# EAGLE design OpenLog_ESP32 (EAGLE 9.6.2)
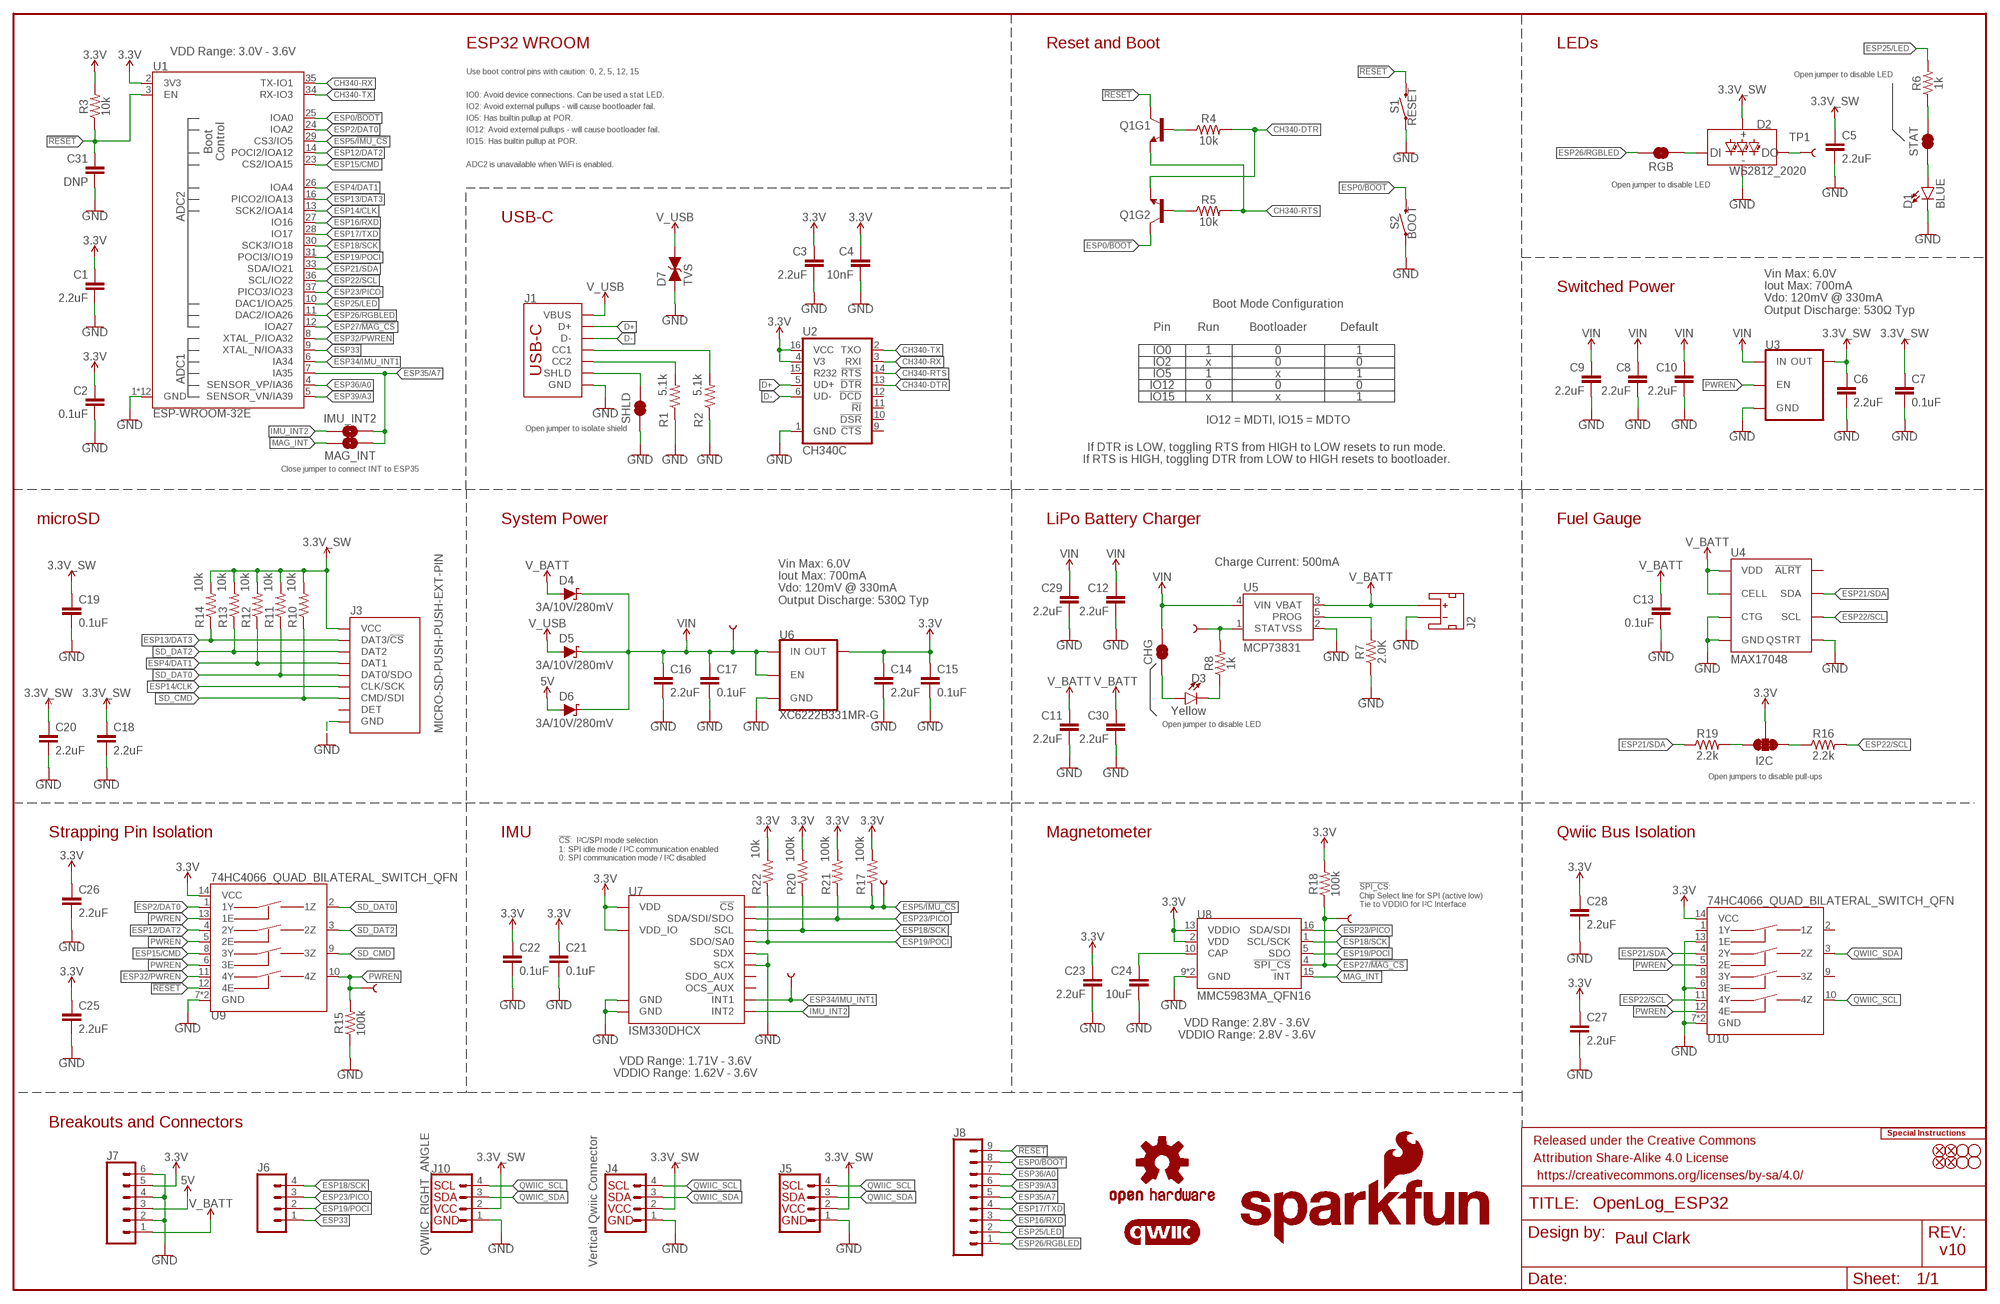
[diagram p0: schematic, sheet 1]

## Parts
C1  2.2uF  2.2UF-0402_TIGHT-10V-10%-X5R  [0402-TIGHT]
C2  0.1uF  0.1UF-0402T-6.3V-10%-X7R  [0402-TIGHT]
C3  2.2uF  2.2UF-0402_TIGHT-10V-10%-X5R  [0402-TIGHT]
C4  10nF  10NF-0402T-25V-10%-X7R-WE  [0402-TIGHT]
C5  2.2uF  2.2UF-0402_TIGHT-10V-10%-X5R  [0402-TIGHT]
C6  2.2uF  2.2UF-0402_TIGHT-10V-10%-X5R  [0402-TIGHT]
C7  0.1uF  0.1UF-0402T-6.3V-10%-X7R  [0402-TIGHT]
C8  2.2uF  2.2UF-0402_TIGHT-10V-10%-X5R  [0402-TIGHT]
C9  2.2uF  2.2UF-0402_TIGHT-10V-10%-X5R  [0402-TIGHT]
C10  2.2uF  2.2UF-0402_TIGHT-10V-10%-X5R  [0402-TIGHT]
C11  2.2uF  2.2UF-0402_TIGHT-10V-10%-X5R  [0402-TIGHT]
C12  2.2uF  2.2UF-0402_TIGHT-10V-10%-X5R  [0402-TIGHT]
C13  0.1uF  0.1UF-0402T-6.3V-10%-X7R  [0402-TIGHT]
C14  2.2uF  2.2UF-0402_TIGHT-10V-10%-X5R  [0402-TIGHT]
C15  0.1uF  0.1UF-0402T-6.3V-10%-X7R  [0402-TIGHT]
C16  2.2uF  2.2UF-0402_TIGHT-10V-10%-X5R  [0402-TIGHT]
C17  0.1uF  0.1UF-0402T-6.3V-10%-X7R  [0402-TIGHT]
C18  2.2uF  2.2UF-0402_TIGHT-10V-10%-X5R  [0402-TIGHT]
C19  0.1uF  0.1UF-0402T-6.3V-10%-X7R  [0402-TIGHT]
C20  2.2uF  2.2UF-0402_TIGHT-10V-10%-X5R  [0402-TIGHT]
C21  0.1uF  0.1UF-0402T-6.3V-10%-X7R  [0402-TIGHT]
C22  0.1uF  0.1UF-0402T-6.3V-10%-X7R  [0402-TIGHT]
C23  2.2uF  2.2UF-0402_TIGHT-10V-10%-X5R  [0402-TIGHT]
C24  10uF  10UF-0402T-6.3V-20%  [0402-TIGHT]
C25  2.2uF  2.2UF-0402_TIGHT-10V-10%-X5R  [0402-TIGHT]
C26  2.2uF  2.2UF-0402_TIGHT-10V-10%-X5R  [0402-TIGHT]
C27  2.2uF  2.2UF-0402_TIGHT-10V-10%-X5R  [0402-TIGHT]
C28  2.2uF  2.2UF-0402_TIGHT-10V-10%-X5R  [0402-TIGHT]
C29  2.2uF  2.2UF-0402_TIGHT-10V-10%-X5R  [0402-TIGHT]
C30  2.2uF  2.2UF-0402_TIGHT-10V-10%-X5R  [0402-TIGHT]
C31  DNP  DNP-0402-TIGHT_NO_CREAM  [0402-TIGHT_NO_CREAM]
CHG  JUMPER-SMT_2_NC_TRACE_SILK  [SMT-JUMPER_2_NC_TRACE_SILK]
D1  BLUE  LED-BLUE0603  [LED-0603]
D2  WS2812_2020  [WS2812-2020]
D3  Yellow  LED-YELLOW0603  [LED-0603]
D4  3A/10V/280mV  DIODE-SCHOTTKY-BAT60A  [SOD-323]
D5  3A/10V/280mV  DIODE-SCHOTTKY-BAT60A  [SOD-323]
D6  3A/10V/280mV  DIODE-SCHOTTKY-BAT60A  [SOD-323]
D7  TVS  DIODE_TVS  [0603]
FD1  FIDUCIAL1X2  [FIDUCIAL-1X2]
FD2  FIDUCIAL1X2  [FIDUCIAL-1X2]
FD3  FIDUCIAL1X2  [FIDUCIAL-1X2]
FD4  FIDUCIAL1X2  [FIDUCIAL-1X2]
FRAME1  FRAME-LEDGER  [CREATIVE_COMMONS]
H1  STAND-OFFTIGHT  [STAND-OFF-TIGHT]
H2  STAND-OFFTIGHT  [STAND-OFF-TIGHT]
H3  STAND-OFFTIGHT  [STAND-OFF-TIGHT]
H4  STAND-OFFTIGHT  [STAND-OFF-TIGHT]
I2C  JUMPER-SMT_3_2-NC_TRACE_SILK  [SMT-JUMPER_3_2-NC_TRACE_SILK]
IMU_!CS!  TEST-POINT3X5  [PAD.03X.05]
IMU_INT1  TEST-POINT3X5  [PAD.03X.05]
IMU_INT2  JUMPER-SMT_2_NO_SILK  [SMT-JUMPER_2_NO_SILK]
J1  USB_C_4-LAYER_PADS  [USB-C-16P_4LAYER-PADS]
J2  JST_2MM_MALE  [JST-2-SMD]
J3  MICRO-SD-PUSH-PUSH-EXT-PIN  [MICROSD-EXTERNALPIN]
J4  Vertical Qwiic Connector  QWIIC_CONNECTOR  [JST04_1MM_VERT]
J5  I2C_STANDARD_NO_SILK  [1X04_NO_SILK]
J6  CONN_041X04_NO_SILK_NO_POP  [1X04_NO_SILK]
J7  CONN_06NO_SILK_NO_POP  [1X06_NO_SILK]
J8  CONN_09NO_SILK  [1X09_NO_SILK]
J10  QWIIC_RIGHT_ANGLE  QWIIC_CONNECTORJS-1MM  [JST04_1MM_RA]
LOGO1  SPECIAL_INSTRUCTIONS-ORDERING  [ORDERING_INSTRUCTIONS]
LOGO3  QWIIC_LOGO_6MM  [QWIIC_6MM]
LOGO4  OSHW-LOGOS  [OSHW-LOGO-S]
LOGO5  SFE_LOGO_NAME.2_INCH  [SFE_LOGO_NAME_.2]
LOGO6  SFE_LOGO_FLAME.2_INCH  [SFE_LOGO_FLAME_.2]
MAG_!CS!  TEST-POINT3X5  [PAD.03X.05]
MAG_INT  JUMPER-SMT_2_NO_SILK  [SMT-JUMPER_2_NO_SILK]
PWREN  TEST-POINT3X5  [PAD.03X.05]
Q1  TRANS_NPN_DUAL-MBT3904DW1T1  [SC70-6]
R1  5.1k  5.1KOHM-0402T-1/16W-1%  [0402-TIGHT]
R2  5.1k  5.1KOHM-0402T-1/16W-1%  [0402-TIGHT]
R3  10k  10KOHM-0402T-1/16W-1%  [0402-TIGHT]
R4  10k  10KOHM-0402T-1/16W-1%  [0402-TIGHT]
R5  10k  10KOHM-0402T-1/16W-1%  [0402-TIGHT]
R6  1k  1KOHM-0402T-1/16W-1%  [0402-TIGHT]
R7  2.0K  2.0KOHM-0402T-1/16W-1%  [0402-TIGHT]
R8  1k  1KOHM-0402T-1/16W-1%  [0402-TIGHT]
R10  10k  10KOHM-0402T-1/16W-1%  [0402-TIGHT]
R11  10k  10KOHM-0402T-1/16W-1%  [0402-TIGHT]
R12  10k  10KOHM-0402T-1/16W-1%  [0402-TIGHT]
R13  10k  10KOHM-0402T-1/16W-1%  [0402-TIGHT]
R14  10k  10KOHM-0402T-1/16W-1%  [0402-TIGHT]
R15  100k  100KOHM-0402T-1/16W-1%  [0402-TIGHT]
R16  2.2k  2.2KOHM-0402T-1/16W-1%  [0402-TIGHT]
R17  100k  100KOHM-0402T-1/16W-1%  [0402-TIGHT]
R18  100k  100KOHM-0402T-1/16W-1%  [0402-TIGHT]
R19  2.2k  2.2KOHM-0402T-1/16W-1%  [0402-TIGHT]
R20  100k  100KOHM-0402T-1/16W-1%  [0402-TIGHT]
R21  100k  100KOHM-0402T-1/16W-1%  [0402-TIGHT]
R22  10k  10KOHM-0402T-1/16W-1%  [0402-TIGHT]
RGB  JUMPER-SMT_2_NC_TRACE_SILK  [SMT-JUMPER_2_NC_TRACE_SILK]
S1  RESET  MOMENTARY-SWITCH-SPST-SMD-RIGHT-ANGLE  [TACTILE_SWITCH_SMD_RIGHT_ANGLE]
S2  BOOT  MOMENTARY-SWITCH-SPST-SMD-RIGHT-ANGLE  [TACTILE_SWITCH_SMD_RIGHT_ANGLE]
SHLD  JUMPER-SMT_2_NC_TRACE_SILK  [SMT-JUMPER_2_NC_TRACE_SILK]
STAT  JUMPER-SMT_2_NC_TRACE_SILK  [SMT-JUMPER_2_NC_TRACE_SILK]
TP1  TEST-POINT3X5  [PAD.03X.05]
U1  ESP-WROOM-32E  ESP-WROOM-3232D-NARROW  [ESP-WROOM-32D-NARROW]
U2  CH340C  [SO016]
U3  XC6222B331MR-G  [SOT23-5]
U4  MAX17048  MAX17048DFN8  [DFN-8]
U5  MCP73831  [SOT23-5]
U6  XC6222B331MR-G  [SOT23-5]
U7  ISM330DHCX  [LGA-14L]
U8  MMC5983MA_QFN16  [LGA-16-3X3MM-4X4PINS]
U9  74HC4066_QUAD_BILATERAL_SWITCH_QFN  [14-QFN]
U10  74HC4066_QUAD_BILATERAL_SWITCH_QFN  [14-QFN]
VIN  TEST-POINT3X5  [PAD.03X.05]
VIN1  TEST-POINT3X5  [PAD.03X.05]

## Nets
3.3V: C1.1 C2.1 C3.1 C4.1 C14.1 C15.1 C21.1 C22.1 C23.1 C25.1 C26.1 C27.1 C28.1 I2C.2 J7.5 R3.2 R17.2 R18.2 R20.2 R21.2 R22.2 U1.2(3V3) U2.4(V3) U2.16(VCC) U6.5(OUT) U7.P5(VDD_IO) U7.P8(VDD) U8.2(VDD) U8.13(VDDIO) U9.14(VCC) U10.14(VCC)
3.3V_SW: C5.1 C6.1 C7.1 C18.1 C19.1 C20.1 D2.VCC J3.4(VCC) J4.2 J5.2 J10.2 R10.2 R11.2 R12.2 R13.2 R14.2 U3.5(OUT)
5V: D6.A J7.3
!RESET!: C31.1 J8.9 Q1.3(C) R3.1 S1.2 U1.3(EN) U9.12(4E)
CAP: C24.1 U8.10(CAP)
CH340-DTR: Q1.1(E) R4.2 U2.13(!DTR)
CH340-RTS: Q1.4(E) R5.2 U2.14(!RTS)
CH340-RX: U1.35(TX-IO1) U2.3(RXI)
CH340-TX: U1.34(RX-IO3) U2.2(TXO)
D+: J1.A6(D+) J1.B6(D+) U2.5(UD+)
D-: J1.A7(D-) J1.B7(D-) U2.6(UD-)
ESP0/!BOOT!: J8.8 Q1.6(C) S2.2 U1.25(IOA0)
ESP2/DAT0: U1.24(IOA2) U9.1(1Y)
ESP4/DAT1: J3.8(DAT1) R12.1 U1.26(IOA4)
ESP5/!IMU_CS!: IMU_!CS!.1 R17.1 U1.29(CS3/IO5) U7.P12(!CS!)
ESP12/DAT2: U1.14(POCI2/IOA12) U9.4(2Y)
ESP13/DAT3: J3.2(DAT3/!CS!) R14.1 U1.16(PICO2/IOA13)
ESP14/CLK: J3.5(CLK/SCK) U1.13(SCK2/IOA14)
ESP15/CMD: U1.23(CS2/IOA15) U9.8(3Y)
ESP16/RXD: J8.3 U1.27(IO16)
ESP17/TXD: J8.4 U1.28(IO17)
ESP18/SCK: J6.4 R20.1 U1.30(SCK3/IO18) U7.P13(SCL) U8.1(SCL/SCK)
ESP19/POCI: J6.2 R22.1 U1.31(POCI3/IO19) U7.P1(SDO/SA0) U8.5(SDO)
ESP21/SDA: R19.1 U1.33(SDA/IO21) U4.8(SDA) U10.4(2Y)
ESP22/SCL: R16.2 U1.36(SCL/IO22) U4.7(SCL) U10.11(4Y)
ESP23/PICO: J6.3 R21.1 U1.37(PICO3/IO23) U7.P14(SDA/SDI/SDO) U8.16(SDA/SDI)
ESP25/LED: J8.2 R6.2 U1.10(DAC1/IOA25)
ESP26/RGBLED: J8.1 RGB.2 U1.11(DAC2/IOA26)
ESP27/!MAG_CS!: MAG_!CS!.1 R18.1 U1.12(IOA27) U8.4(!SPI_CS!)
ESP32/PWREN: U1.8(XTAL_P/IOA32) U9.11(4Y)
ESP33: J6.1 U1.9(XTAL_N/IOA33)
ESP34/IMU_INT1: IMU_INT1.1 U1.6(IA34) U7.P4(INT1)
ESP35/A7: IMU_INT2.2 J8.5 MAG_INT.2 U1.7(IA35)
ESP36/A0: J8.7 U1.4(SENSOR_VP/IA36)
ESP39/A3: J8.6 U1.5(SENSOR_VN/IA39)
GND: C1.2 C2.2 C3.2 C4.2 C5.2 C6.2 C7.2 C8.2 C9.2 C10.2 C11.2 C12.2 C13.2 C14.2 C15.2 C16.2 C17.2 C18.2 C19.2 C20.2 C21.2 C22.2 C23.2 C24.2 C25.2 C26.2 C27.2 C28.2 C29.2 C30.2 C31.2 D1.C D2.GND D7.1(A) J1.GND J1.GND2(GND) J2.1(-) J3.6(GND) J3.10(GND) J3.11(GND) J3.12(GND) J3.13(GND) J4.1 J5.1 J7.2 J7.4 J7.6 J10.1 R1.1 R2.1 R7.1 R15.1 S1.1 S2.1 SHLD.1 U1.1(GND) U1.15(GND) U1.38(GND) U1.GND1(GND) U1.GNDT1(GND) U1.GNDT2(GND) U1.GNDT3(GND) U1.GNDT4(GND) U1.GNDT5(GND) U1.GNDT6(GND) U1.GNDT7(GND) U1.GNDT8(GND) U2.1(GND) U3.2(GND) U4.1(CTG) U4.4(GND) U4.6(QSTRT) U4.9(GND) U5.2(VSS) U6.2(GND) U7.P2(SDX) U7.P3(SCX) U7.P6(GND) U7.P7(GND) U8.9(GND) U8.11(GND) U9.7(GND) U9.EPAD(GND) U10.6(3E) U10.7(GND) U10.13(1E) U10.EPAD(GND)
IMU_INT2: IMU_INT2.1 U7.P9(INT2)
MAG_INT: MAG_INT.1 U8.15(INT)
N$1: J1.B5(CC2) R1.2
N$2: J1.A5(CC1) R2.2
N$4: Q1.2(B) R5.1
N$5: Q1.5(B) R4.1
N$6: R6.1 STAT.2
N$7: D2.DO TP1.1
N$8: CHG.1 D3.A
N$9: D3.C R8.1
N$10: R8.2 U5.1(STAT) VIN1.1
N$11: R7.2 U5.5(PROG)
N$12: D2.DI RGB.1
N$13: D1.A STAT.1
N$16: I2C.1 R16.1
N$17: I2C.3 R19.2
PWREN: PWREN.1 R15.2 U3.3(EN) U9.5(2E) U9.6(3E) U9.10(4Z) U9.13(1E) U10.5(2E) U10.12(4E)
QWIIC_SCL: J4.4 J5.4 J10.4 U10.10(4Z)
QWIIC_SDA: J4.3 J5.3 J10.3 U10.3(2Z)
SD_CMD: J3.3(CMD/SDI) R10.1 U9.9(3Z)
SD_DAT0: J3.7(DAT0/SDO) R11.1 U9.2(1Z)
SD_DAT2: J3.1(DAT2) R13.1 U9.3(2Z)
SHIELD: J1.SHLD1(SHLD) J1.SHLD2(SHLD) J1.SHLD3(SHLD) J1.SHLD4(SHLD) SHLD.2
V_BATT: C11.1 C13.1 C30.1 D4.A J2.2(+) J7.1 U4.2(CELL) U4.3(VDD) U5.3(VBAT)
V_USB: D5.A D7.2(C) J1.VBUS1(VBUS) J1.VBUS2(VBUS)
VIN: C8.1 C9.1 C10.1 C12.1 C16.1 C17.1 C29.1 CHG.2 D4.C D5.C D6.C U3.1(IN) U5.4(VIN) U6.1(IN) U6.3(EN) VIN.1
Unconnected: J2.NC1(PAD1) J2.NC2(PAD2) J3.9(DET) U2.9(!CTS) U2.10(!DSR) U2.11(!RI) U2.12(!DCD) U2.15(R232) U4.5(!ALRT) U7.P10(OCS_AUX) U7.P11(SDO_AUX) U10.1(1Y) U10.2(1Z) U10.8(3Y) U10.9(3Z)

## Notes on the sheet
- VDD Range: 3.0V - 3.6V | ESP32 WROOM | Reset and Boot | LEDs
- Use boot control pins with caution: 0, 2, 5, 12, 15
- Open jumper to disable LED
- IO0: Avoid device connections. Can be used a stat LED.
- IO2: Avoid external pullups - will cause bootloader fail.
- IO5: Has builtin pullup at POR.
- IO12: Avoid external pullups - will cause bootloader fail.
- IO15: Has builtin pullup at POR.
- ADC2 is unavailable when WiFi is enabled.
- Open jumper to disable LED
- USB-C
- Switched Power
- Boot Mode Configuration
- Vin Max: 6.0V
  Iout Max: 700mA
  Vdo: 120mV @ 330mA
  Output Discharge: 530Ω Typ
- Pin | Run | Bootloader | Default
- IO0 | 1 | 0 | 1
- IO2 | x | 0 | 0
- IO5 | 1 | x | 1
- IO12 | 0 | 0 | 0
- IO15 | x | x | 1
- IO12 = MDTI, IO15 = MDTO
- Open jumper to isolate shield
- If DTR is LOW, toggling RTS from HIGH to LOW resets to run mode.
  If RTS is HIGH, toggling DTR from LOW to HIGH resets to bootloader.
- Close jumper to connect INT to ESP35
- microSD | System Power | LiPo Battery Charger | Fuel Gauge
- Charge Current: 500mA
- Vin Max: 6.0V
  Iout Max: 700mA
  Vdo: 120mV @ 330mA
  Output Discharge: 530Ω Typ
- Open jumper to disable LED
- Open jumpers to disable pull-ups
- Strapping Pin Isolation | IMU | Magnetometer | Qwiic Bus Isolation
- !CS!:  I²C/SPI mode selection
  1: SPI idle mode / I²C communication enabled
  0: SPI communication mode / I²C disabled
- !SPI_CS!:
  Chip Select line for SPI (active low) 
  Tie to VDDIO for I²C Interface
- VDD Range: 2.8V - 3.6V
  VDDIO Range: 2.8V - 3.6V
- VDD Range: 1.71V - 3.6V
  VDDIO Range: 1.62V - 3.6V
- Breakouts and Connectors
- Paul Clark
- v10

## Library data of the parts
C1 C3 C5 C6 C8-C12 C14 C16 C18 C20 C23 C25-C30 = SparkFun-Capacitors:2.2UF: 2.2µF ceramic capacitors; PROD_ID: CAP-14232
C2 C7 C13 C15 C17 C19 C21 C22 = SparkFun-Capacitors:0.1UF: 0.1µF ceramic capacitors; PROD_ID: CAP-14993
C4 = SparkFun-Capacitors:10NF: 0.01uF/10nF/10,000pF ceramic capacitors; PROD_ID: CAP-16508
C24 = SparkFun-Capacitors:10UF: 10.0µF ceramic capacitors; PROD_ID: CAP-14848
C31 = SparkFun-Capacitors:DNP: Do-Not-Populate capacitor
CHG RGB SHLD STAT = SparkFun-Jumpers:JUMPER-SMT_2_NC_TRACE: Normally closed trace jumper
D1 = SparkFun-LED:LED-BLUE: Blue SMD LED; PROD_ID: DIO-08575
D2 = SparkFun-LED:WS2812: Addressable RGB LED - 1 Wire Common names: WS2812, SK6812, Neopixel, APA-106, etc. SMD LED with built-in controller IC. Color: Red/Green/Blue SparkFun Products: LED-SMD RGB (WS2812) LED - RGB Addressable, PTH, 5mm Diffused (5 Pack) LED - RGB Addressable, PTH, 5mm Clear (5 Pack) Blynk Board -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; PROD_ID: DIO-15591
D3 = SparkFun-LED:LED-YELLOW: Yellow SMD LED; PROD_ID: DIO-09003
D4-D6 = SparkFun-DiscreteSemi:DIODE-SCHOTTKY: Schottky diode; PROD_ID: DIO-14072
D7 = SparkFun-DiscreteSemi:DIODE_TVS; PROD_ID: DIO-14502; VALUE: 24V
FD1-FD4 = SparkFun-Aesthetics:FIDUCIAL: Fiducial Alignment Points
FRAME1 = SparkFun-Aesthetics:FRAME-LEDGER: Schematic Frame - Ledger
H1-H4 = SparkFun-Hardware:STAND-OFF: Stand Off
I2C = SparkFun-Jumpers:JUMPER-SMT_3_2-NC_TRACE: Normally closed trace jumper (2 of 2 connections) This jumper has a trace between all three pads so they are normally closed (NC). Use a razor knife to open the connection(s). For best results follow the IPC guidelines for cutting traces: Cutout at least 0.063 mm (0.005 in). Remove all loose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
IMU_!CS! IMU_INT1 MAG_!CS! PWREN TP1 VIN VIN1 = SparkFun-Connectors:TEST-POINT: SparkFun Test Points
IMU_INT2 MAG_INT = SparkFun-Jumpers:JUMPER-SMT_2_NO: Normally open jumper
J1 = SparkFun-Connectors:USB_C: USB Type C 16Pin Connector Super Speed pins not available on the 16-pin purely SMD connector so this part is best for USB 2.0 implementations. D1 and D2 are tied together enabling D+/- no matter which way the cable is plugged into the connector. The two channel configuration pins (CC1/2) are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; PROD_ID: CONN-14122
J2 = SparkFun-Connectors:JST_2MM_MALE: JST 2MM MALE RA CONNECTOR Two pin, compact surface mount connector. Commonly used as a battery input connection point. We really like the solid locking feeling and high current rating on these small connectors. We use these all the time as battery connectors. Mates to single-cell LiPo batteries.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; PROD_ID: CONN-11443; SF_ID: PRT-08612
J3 = SparkFun-Connectors:MICRO-SD: microSD Socket for Transflash Various sockets for µSD. tDoc lines correctly indicate media card edge positions when inserting (unlocked, locked, depressed). NOTE: CD1 and CD2 are connected internally, and the default detect state of the socket is detect pin to ground. SparkFun Products: WAV Trigger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; PROD_ID: CONN-16110
J4 = SparkFun-Connectors:QWIIC_CONNECTOR: SparkFun I2C Standard Qwiic Connector An SMD 1mm pitch JST connector makes it easy and quick (get it? Qwiic?) to connect I2C devices to each other. The Qwiic system enables fast and solderless connection between popular platforms and various sensors and actuators. We carry 200mm, 100mm, 50mm, and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; PROD_ID: CONN-14483
J5 = SparkFun-Connectors:I2C_STANDARD: SparkFun I2C Standard Pinout Header SparkFun has standardized on a pinout for all I2C based sensor breakouts. This pinout allows I2C boards to be plugged directly into the headers on Arduino Uno compatible boards, and to be daisy chained easily. Example SparkFun Products: SparkFun Atmospheric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
J6 = SparkFun-Connectors:CONN_04: Multi connection point. Often used as Generic Header-pin footprint for 0.1 inch spaced/style header connections On any of the 0.1 inch spaced packages, you can populate with these: Break Away Headers - Straight (PRT-00116) Break Away Male Headers - Right Angle (PRT-00553) Female Headers (PRT-00115)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
J7 = SparkFun-Connectors:CONN_06: Multi connection point. Often used as Generic Header-pin footprint for 0.1 inch spaced/style header connections On any of the 0.1 inch spaced packages, you can populate with these: Break Away Headers - Straight (PRT-00116) Break Away Male Headers - Right Angle (PRT-00553) Female Headers (PRT-00115)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
J8 = SparkFun-Connectors:CONN_09: Multi connection point. Often used as Generic Header-pin footprint for 0.1 inch spaced/style header connections On any of the 0.1 inch spaced packages, you can populate with these: Break Away Headers - Straight (PRT-00116) Break Away Male Headers - Right Angle (PRT-00553) Female Headers (PRT-00115)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
J10 = SparkFun-Connectors:QWIIC_CONNECTOR: SparkFun I2C Standard Qwiic Connector An SMD 1mm pitch JST connector makes it easy and quick (get it? Qwiic?) to connect I2C devices to each other. The Qwiic system enables fast and solderless connection between popular platforms and various sensors and actuators. We carry 200mm, 100mm, 50mm, and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; PROD_ID: CONN-13694
LOGO1 = SparkFun-Aesthetics:SPECIAL_INSTRUCTIONS: Special Ordering/Production Instructions Alert
LOGO3 = SparkFun-Aesthetics:QWIIC_LOGO: Qwiic Logos for placement on schematic and PCB. The 5.5mm silk logo is best for placing next to Qwiic connector.
LOGO4 = SparkFun-Aesthetics:OSHW-LOGO: Open-Source Hardware (OSHW) Logo
LOGO5 = SparkFun-Aesthetics:SFE_LOGO_NAME: SparkFun Font Logo
LOGO6 = SparkFun-Aesthetics:SFE_LOGO_FLAME: SparkFun Flame Logo
Q1 = SparkFun-DiscreteSemi:TRANS_NPN_DUAL: Dual NPN Transistors in Single Package The MBT3904W1 puts two general purpose 3904 NPN transistors in a single package. Datasheet SparkFun Products: SparkFun ESP32 Thing; PROD_ID: TRANS-13337
R1 R2 = SparkFun-Resistors:5.1KOHM; PROD_ID: RES-14340
R3-R5 R10-R14 R22 = SparkFun-Resistors:10KOHM: 10kΩ resistor; PROD_ID: RES-14241
R6 R8 = SparkFun-Resistors:1KOHM: 1kΩ resistor; PROD_ID: RES-14342
R7 = SparkFun-Resistors:2.0KOHM: 2kΩ resistor; PROD_ID: RES-15406
R15 R17 R18 R20 R21 = SparkFun-Resistors:100KOHM: 100kΩ resistor; PROD_ID: RES-13495
R16 R19 = SparkFun-Resistors:2.2KOHM: 2.2kΩ resistor; PROD_ID: RES-14341
S1 S2 = SparkFun-Switches:MOMENTARY-SWITCH-SPST: Momentary Switch (Pushbutton) - SPST; PROD_ID: COMP-12265
U1 = SparkFun-RF:ESP-WROOM-32: ESP-WROOM-32D - trace antenna (includes keepout) ESP-WROOM-32U - U.FL antenna connector Includes both "standard" footprints and "narrow" version (for use with tighter layouts).; PROD_ID: IC-15676
U2 = SparkFun-IC-Comms:CH340C; PROD_ID: IC-14038
U3 U6 = SparkFun-IC-Power:XC6222; IOUT: 700mA; PROD_ID: VREG-16775; VOUT: 3.3V
U4 = SparkFun-IC-Power:MAX17048: Micropower 1-Cell Li+ ModelGauge SparkFun Products Qduino Mini (DEV-13614); PROD_ID: IC-12551
U5 = SparkFun-IC-Power:MCP73831: MCP73831T Li-Ion, Li-Pol Controller Miniature single cell, fully integrated Li-Ion, Li-polymer charge management controller Datasheet SparkFun Products: SparkFun ESP32 Thing SparkFun 9DoF Razor IMU M0; PROD_ID: IC-09995
U7 = SparkFun-Sensors:ISM330DHCX: ISM330DHCX 6DoF The ISM330DHCX is a system-in-package featuring a high-performance 3D digital accelerometer and 3D digital gyroscope tailored for Industry 4.0 applications.; PROD_ID: IC-16693
U8 = SparkFun-Sensors:MMC5983MA: High Performance 3-axis Magnetic Sensor The MMC5983MA is an AEC-Q100 qualified complete 3-axis magnetic sensor with on-chip signal processing and integrated I2C/SPI bus suitable for use in automotive applications. The device can be connected directly to a microprocessor, eliminating the need for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; PROD_ID: IC-16314
U9 U10 = SparkFun-IC-Logic:74HC4066_QUAD_BILATERAL_SWITCH: Nexperia Quad Bilateral Switch The 74HC4066 is a quad single pole, single throw analog switch. Each switch features two input/output terminals (nY and nZ) and an active HIGH enable input (nE). When nE is LOW, the analog switch is turned off. Inputs include clamp diodes. This enables the use of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; PROD_ID: IC-16528

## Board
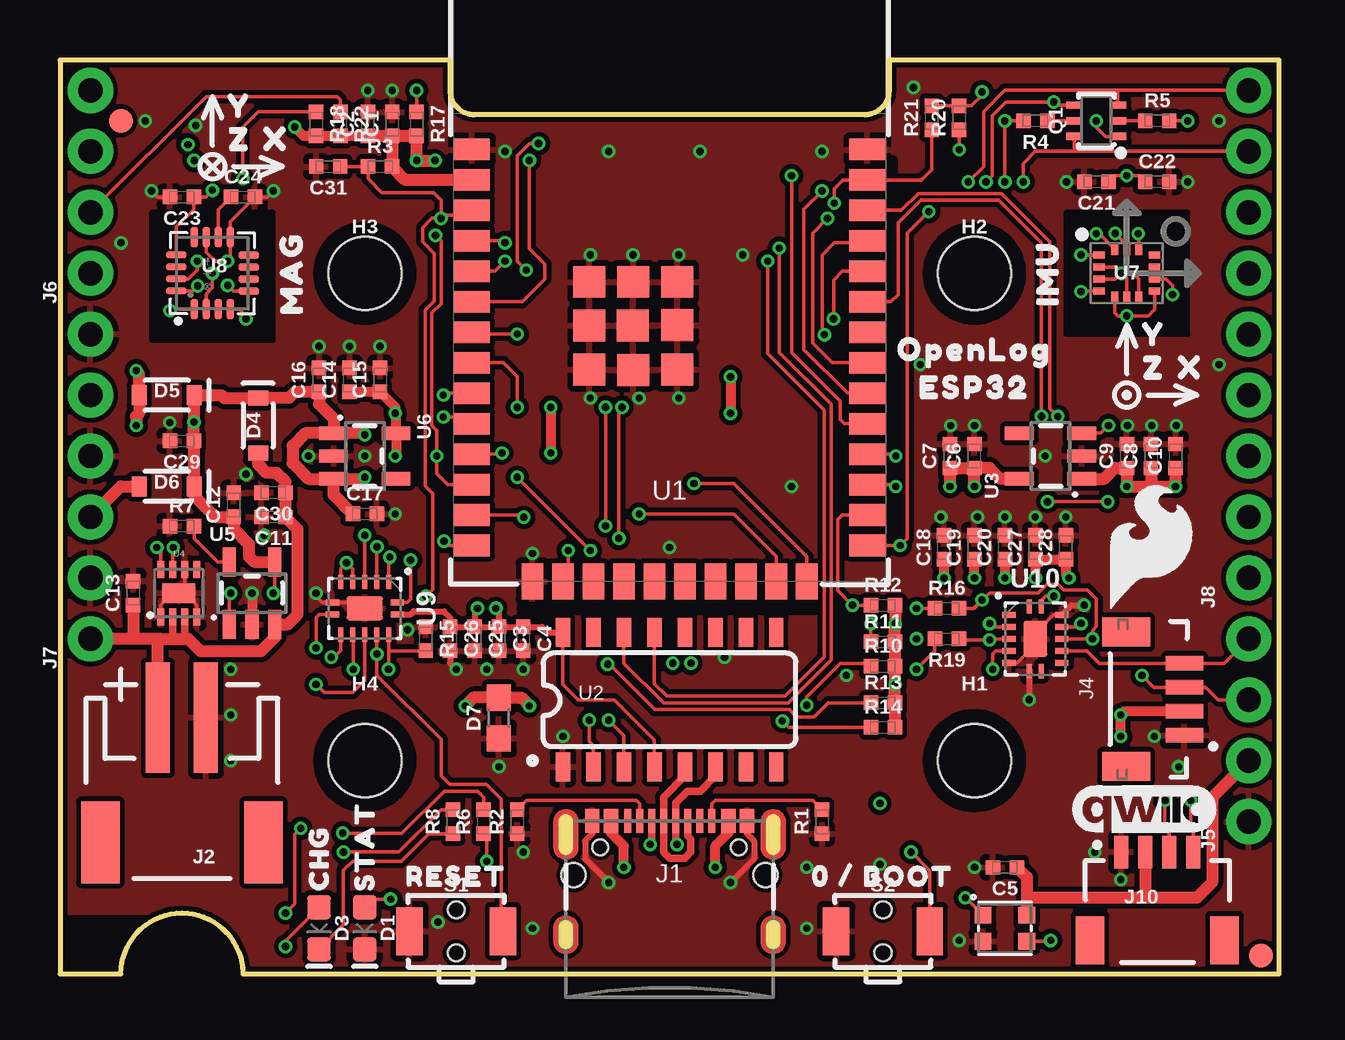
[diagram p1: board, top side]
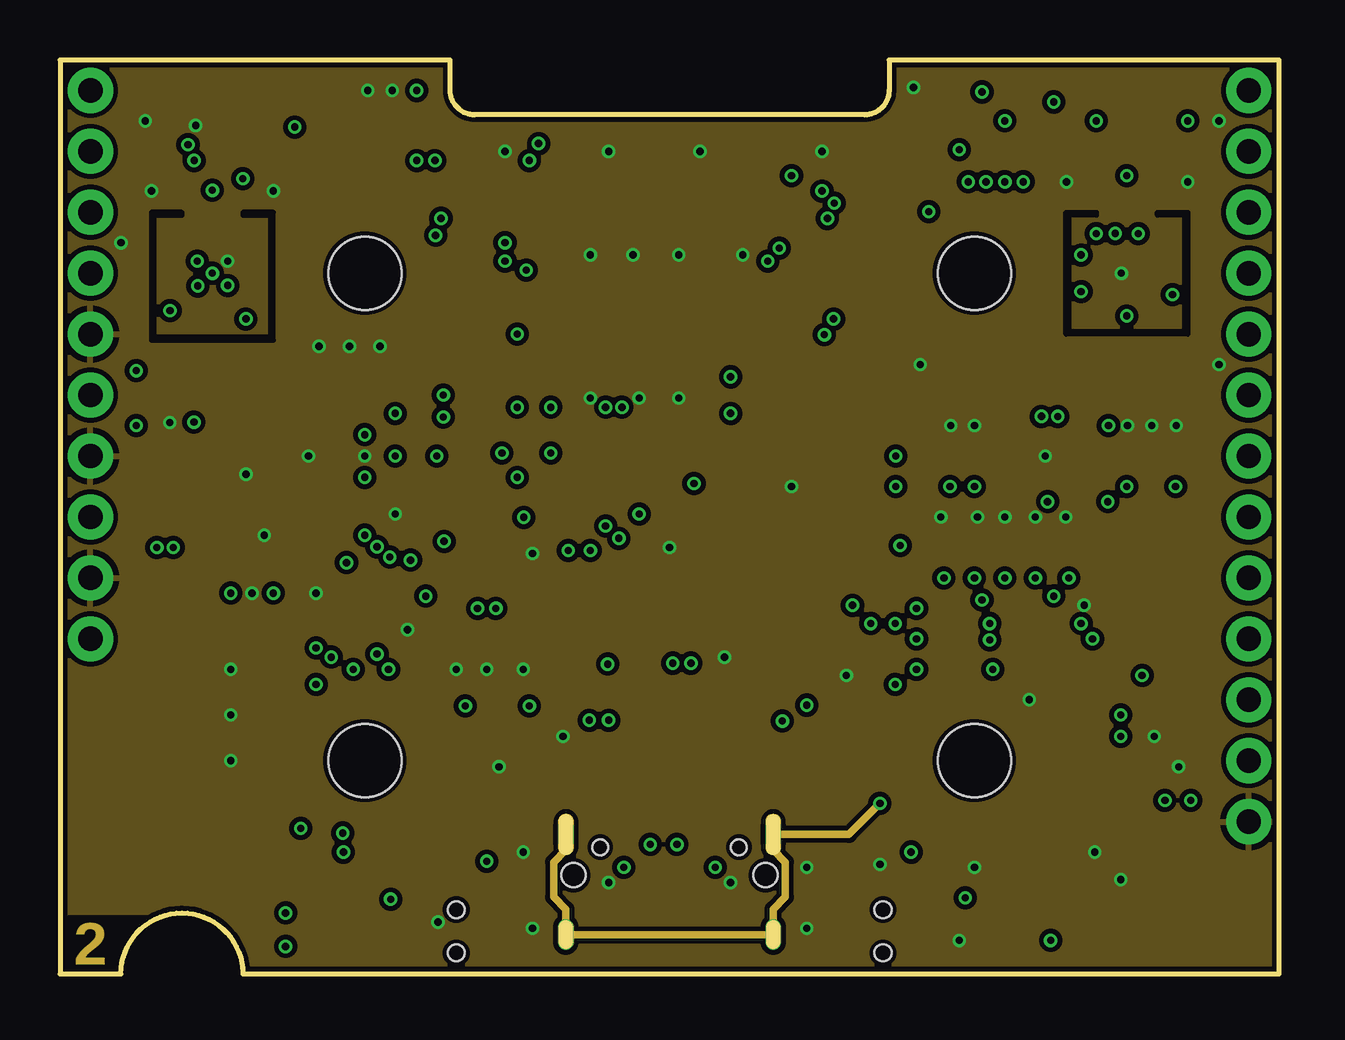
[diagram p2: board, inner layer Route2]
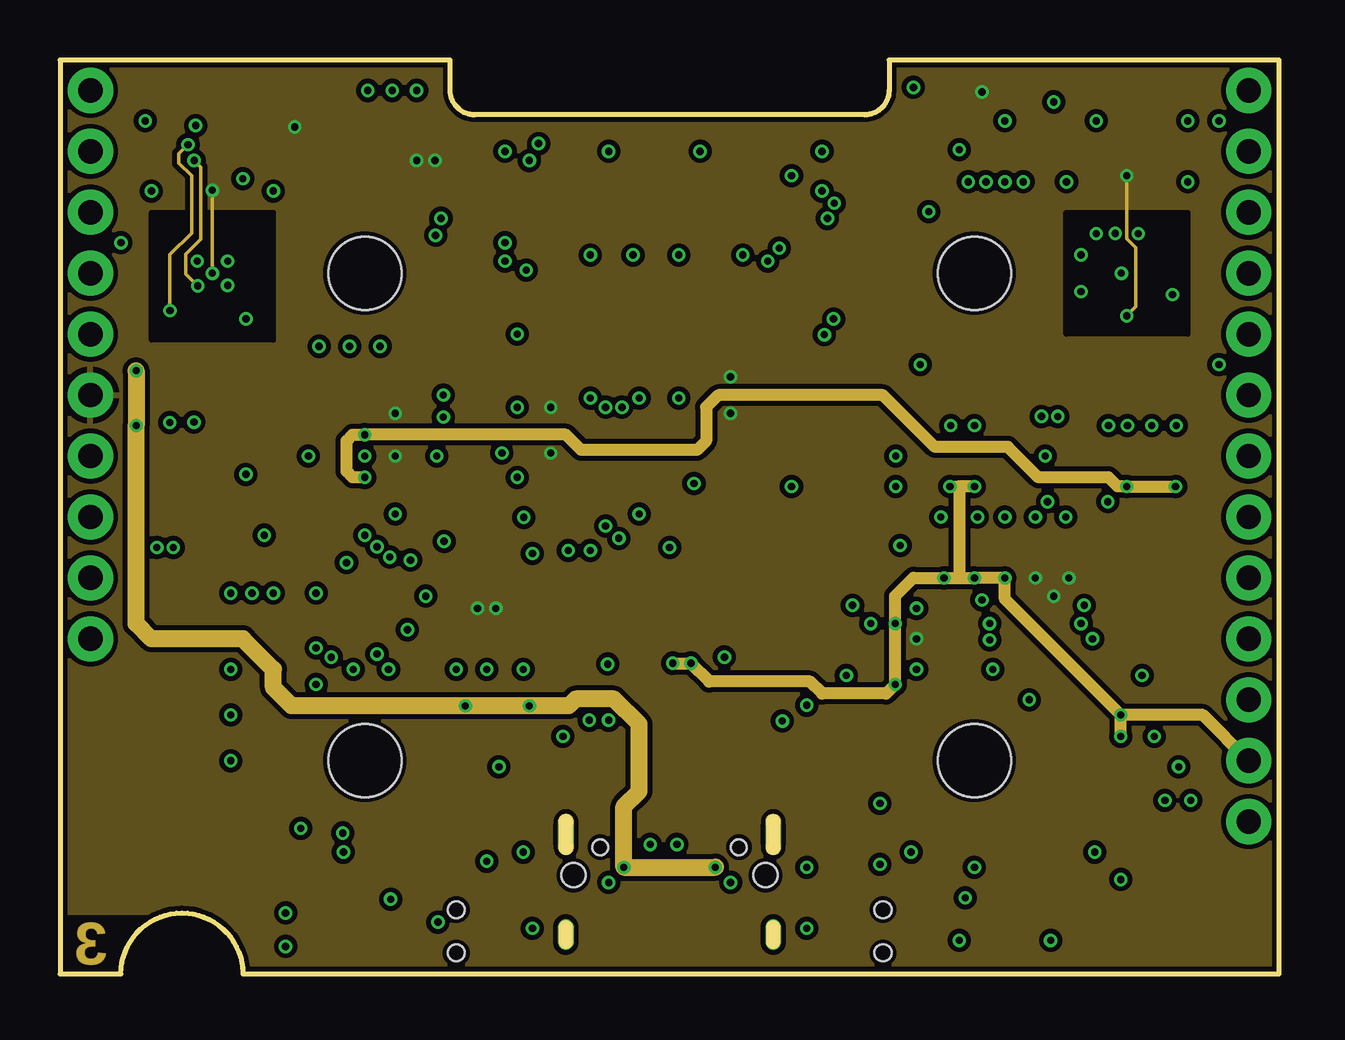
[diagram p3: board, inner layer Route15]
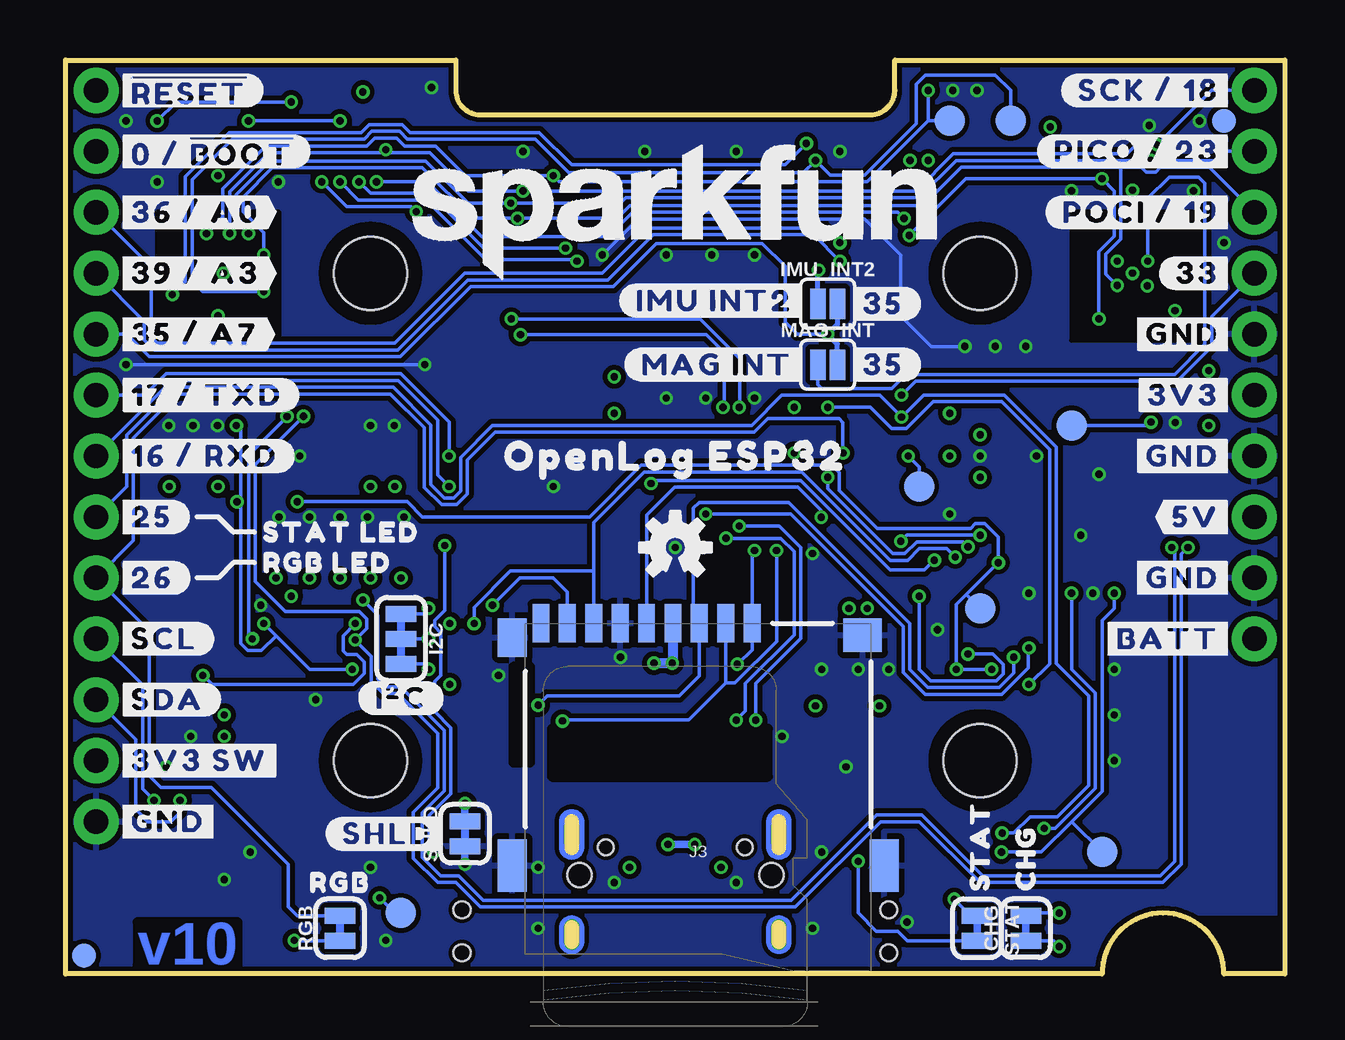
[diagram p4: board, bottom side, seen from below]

Size 50.8 x 38.1 mm. Coordinates in mm from the lower left corner, seen from the top.
Outline: 0,0 2.54,0 arc-90 5.08,2.54 arc-90 7.62,0 50.8,0 50.8,38.1 34.54,38.1 34.54,36.83 arc-90 33.53,35.81 17.27,35.81 arc-90 16.26,36.83 16.26,38.1 0,38.1 0,0
Copper layers (1*2*15*16): Top 0.035559375mm / dielectric 0.47751875mm / Route2 0.035559375mm / dielectric 0.47751875mm / Route15 0.035559375mm / dielectric 0.47751875mm / Bottom 0.035559375mm
Design rules "SparkFun-4-Layer-Minimum-JLCPCB": minimum track width 5mil, minimum drill 0.2mm, track to track 5mil, track to pad 5mil, pad to pad 5mil, via to via 5mil, smd to smd 5mil, copper to edge 7mil, drill to drill 7mil, minimum pad ring 5mil, minimum via ring 5mil, stop-mask expansion 2.5mil, vias tented up to drill 25mil, thermal gap 10mil
tRestrict: 2 lines

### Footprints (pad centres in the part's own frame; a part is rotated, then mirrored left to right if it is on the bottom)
0402-TIGHT = smd 0.6 x 0.6: 1 -0.5,0; 2 0.5,0
0402-TIGHT_NO_CREAM = smd 0.6 x 0.6: 1 -0.5,0; 2 0.5,0
SMT-JUMPER_2_NC_TRACE_SILK = smd 0.66 x 1.27: 1 -0.521,0; 2 0.521,0
LED-0603 = smd 1 x 1: A -0.877,0; C 0.877,0
WS2812-2020 = smd 0.7 x 0.7: DI -0.915,0.55; DO 0.915,-0.55; GND 0.915,0.55; VCC -0.915,-0.55
SOD-323 = smd 0.63 x 0.83: A 1.15,0; C -1.15,0
0603 = smd 1.1 x 1: 1 -0.85,0; 2 0.85,0
FIDUCIAL-1X2 = smd 1 x 1: 1 0,0
STAND-OFF-TIGHT = hole 3.048: 0,0
SMT-JUMPER_3_2-NC_TRACE_SILK = smd 0.66 x 1.27: 1 -1.041,0; 2 0,0; 3 1.041,0
PAD.03X.05 = smd 1.27 x 1.27: 1 0,0
SMT-JUMPER_2_NO_SILK = smd 0.635 x 1.27: 1 -0.406,0; 2 0.406,0
USB-C-16P_4LAYER-PADS = smd 0.3 x 1: A5 -1.25,-0.34; A6 -0.25,-0.34; A7 0.25,-0.34; A8 1.25,-0.34; B5 1.75,-0.34; B6 0.75,-0.34; B7 -0.75,-0.34; B8 -1.75,-0.34 | smd 0.6 x 1: GND -3.225,-0.34; GND2 3.225,-0.34; VBUS1 -2.45,-0.34; VBUS2 2.45,-0.34 | drill 0.4 pad 0.6 long: SHLD1 -4.318,-0.915; SHLD2 4.318,-0.915; SHLD3 -4.318,-5.095; SHLD4 4.318,-5.095 | hole 0.65: -2.89,-1.445; 2.89,-1.445
JST-2-SMD = smd 1 x 4.6: 1 -1,-3.7; 2 1,-3.7 | smd 1.6 x 3.4: NC1 -3.4,1.5; NC2 3.4,1.5
MICROSD-EXTERNALPIN = smd 0.7 x 1.6: 1 2.25,10.5; 2 1.15,10.5; 3 0.05,10.5; 4 -1.05,10.5; 5 -2.15,10.5; 6 -3.25,10.5; 7 -4.35,10.5; 8 -5.45,10.5; 9 -6.55,10.5 | smd 1.2 x 1.6: 10 -7.75,9.9 | smd 1.2 x 2.2: 11 -7.75,0.4; 12 7.75,0.4 | smd 1.6 x 1.4: 13 6.85,10 | hole 1: 3.05,0; -4.95,0
JST04_1MM_VERT = smd 0.6 x 1.55: 1 -1.478,0.775; 2 -0.478,0.775; 3 0.522,0.775; 4 1.522,0.775 | smd 1.2 x 2: NC1 -2.778,3.2; NC2 2.822,3.2
1X04_NO_SILK = drill 1.016 pad 1.88: 1 0,0; 2 2.54,0; 3 5.08,0; 4 7.62,0
1X06_NO_SILK = drill 1.016 pad 1.88: 1 0,0; 2 2.54,0; 3 5.08,0; 4 7.62,0; 5 10.16,0; 6 12.7,0
1X09_NO_SILK = drill 1.016 pad 1.88: 1 0,0; 2 2.54,0; 3 5.08,0; 4 7.62,0; 5 10.16,0; 6 12.7,0; 7 15.24,0; 8 17.78,0; 9 20.32,0
JST04_1MM_RA = smd 0.6 x 1.35: 1 -1.5,0; 2 -0.5,0; 3 0.5,0; 4 1.5,0 | smd 1.2 x 2: NC1 2.8,-3.675; NC2 -2.8,-3.675
SC70-6 = smd 0.3 x 0.66: 1 -0.65,-0.92; 2 0,-0.92; 3 0.65,-0.92; 4 0.65,0.92; 5 0,0.92; 6 -0.65,0.92
TACTILE_SWITCH_SMD_RIGHT_ANGLE = smd 1.1 x 2: 1 -1.95,0; 2 1.95,0 | hole 0.7: 0,0.9; 0,-0.9
ESP-WROOM-32D-NARROW = smd 0.9 x 1.5: 1 6.43,8.238; 2 5.16,8.238; 3 3.89,8.238; 4 2.62,8.238; 5 1.35,8.238; 6 0.08,8.238; 7 -1.19,8.238; 8 -2.46,8.238; 9 -3.73,8.238; 10 -5,8.238; 11 -6.27,8.238; 12 -7.54,8.238; 13 -8.81,8.238; 14 -10.08,8.238; 25 -10.08,-8.238; 26 -8.81,-8.238; 27 -7.54,-8.238; 28 -6.27,-8.238; 29 -5,-8.238; 30 -3.73,-8.238; 31 -2.46,-8.238; 32 -1.19,-8.238; 33 0.08,-8.238; 34 1.35,-8.238; 35 2.62,-8.238; 36 3.89,-8.238; 37 5.16,-8.238; 38 6.43,-8.238 | smd 1.5 x 0.9: 15 -11.57,5.715; 16 -11.57,4.445; 17 -11.57,3.175; 18 -11.57,1.905; 19 -11.57,0.635; 20 -11.57,-0.635; 21 -11.57,-1.905; 22 -11.57,-3.175; 23 -11.57,-4.445; 24 -11.57,-5.715 | smd 1.33 x 1.33: GND1 -0.912,1.531; GNDT1 -2.751,3.346; GNDT2 -2.761,1.516; GNDT3 -2.751,-0.314; GNDT4 -0.891,-0.324; GNDT5 0.909,-0.314; GNDT6 0.909,1.516; GNDT7 0.909,3.346; GNDT8 -0.921,3.346
SO016 = smd 0.6 x 1.2: 1 -4.445,-2.8; 2 -3.175,-2.8; 3 -1.905,-2.8; 4 -0.635,-2.8; 5 0.635,-2.8; 6 1.905,-2.8; 7 3.175,-2.8; 8 4.445,-2.8; 9 4.445,2.8; 10 3.175,2.8; 11 1.905,2.8; 12 0.635,2.8; 13 -0.635,2.8; 14 -1.905,2.8; 15 -3.175,2.8; 16 -4.445,2.8
SOT23-5 = smd 0.55 x 1.2: 1 -0.95,-1.3; 2 0,-1.3; 3 0.95,-1.3; 4 0.95,1.3; 5 -0.95,1.3
DFN-8 = smd 0.3 x 0.7: 1 -0.75,-0.99; 2 -0.25,-0.99; 3 0.25,-0.99; 4 0.75,-0.99; 5 0.75,0.99; 6 0.25,0.99; 7 -0.25,0.99; 8 -0.75,0.99 | smd 1.38 x 0.8: 9 0,0
LGA-14L = smd 0.48 x 0.3: P1 -1.163,0.75; P2 -1.163,0.25; P3 -1.163,-0.25; P4 -1.163,-0.75; P8 1.163,-0.75; P9 1.163,-0.25; P10 1.163,0.25; P11 1.163,0.75 | smd 0.3 x 0.48: P5 -0.5,-1; P6 0,-1; P7 0.5,-1; P12 0.5,1; P13 0,1; P14 -0.5,1
LGA-16-3X3MM-4X4PINS = smd 0.3 x 0.85: 1 0.754,1.498; 2 0.254,1.498; 3 -0.246,1.498; 4 -0.746,1.498; 9 -0.746,-1.506; 10 -0.246,-1.506; 11 0.254,-1.506; 12 0.754,-1.506 | smd 0.85 x 0.3: 5 -1.508,0.746; 6 -1.508,0.246; 7 -1.508,-0.254; 8 -1.508,-0.754; 13 1.496,-0.764; 14 1.496,-0.264; 15 1.496,0.236; 16 1.496,0.736
14-QFN = smd 0.25 x 0.6: 1 -0.25,1.35; 7 -0.25,-1.35; 8 0.25,-1.35; 14 0.25,1.35 | smd 0.6 x 0.25: 2 -1.1,1; 3 -1.1,0.5; 4 -1.1,0; 5 -1.1,-0.5; 6 -1.1,-1; 9 1.1,-1; 10 1.1,-0.5; 11 1.1,0; 12 1.1,0.5; 13 1.1,1 | smd 1 x 1.5: EPAD 0,0

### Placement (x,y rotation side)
C1  13.84,35.43 90 top
C2  12.83,35.43 90 top
C3  18.29,13.97 270 top
C4  19.3,13.97 270 top
C5  39.37,4.45 180 top
C6  38.1,21.59 90 top
C7  37.08,21.59 90 top
C8  45.47,21.59 90 top
C9  44.45,21.59 90 top
C10  46.48,21.59 90 top
C11  8.89,19.05 180 top
C12  7.24,19.56 90 top
C13  3.05,15.88 90 top
C14  12.06,24.77 90 top
C15  13.34,24.77 90 top
C16  10.79,24.77 90 top
C17  12.7,19.18 0 top
C18  36.83,17.78 90 top
C19  38.1,17.78 90 top
C20  39.37,17.78 90 top
C21  43.18,33.02 180 top
C22  45.72,33.02 0 top
C23  5.08,32.38 180 top
C24  7.62,32.38 0 top
C25  17.27,13.97 270 top
C26  16.26,13.97 270 top
C27  40.64,17.78 90 top
C28  41.91,17.78 90 top
C29  5.08,22.23 180 top
C30  8.89,20.07 180 top
C31  11.18,33.66 180 top
CHG  10.79,1.91 90 bottom
D1  12.7,1.91 270 top
D2  39.37,1.91 180 top
D3  10.79,1.91 270 top
D4  8.26,22.86 270 top
D5  4.45,24.13 180 top
D6  4.45,20.32 180 top
D7  18.29,10.67 90 top
FD1  2.54,35.56 0 bottom
FD2  2.54,35.56 0 top
FD3  50.04,0.76 0 bottom
FD4  50.04,0.76 0 top
FRAME1  not placed on the board
H1  38.1,8.89 0 top
H2  38.1,29.21 0 top
H3  12.7,29.21 0 top
H4  12.7,8.89 0 top
I2C  36.83,13.97 270 bottom
IMU_!CS!  13.97,35.56 0 bottom
IMU_INT1  11.43,35.56 0 bottom
IMU_INT2  19.05,27.94 0 bottom
J1  25.4,6.73 0 top
J2  5.08,6.99 180 top
J3  24.45,4.11 0 bottom
J4  47.62,11.43 90 top
J5  49.53,6.35 90 top
J6  1.27,29.21 90 top
J7  1.27,13.97 90 top
J8  49.53,16.51 90 top
J10  45.72,5.08 0 top
LOGO1  not placed on the board
LOGO3  45.21,6.86 0 top
LOGO4  25.4,17.78 0 bottom
LOGO5  25.4,31.75 0 bottom
LOGO6  45.47,17.78 0 top
MAG_!CS!  15.24,20.32 0 bottom
MAG_INT  19.05,25.4 0 bottom
PWREN  12.7,15.24 0 bottom
Q1  43.18,35.56 90 top
R1  31.75,6.35 90 top
R2  19.05,6.35 90 top
R3  13.34,33.66 0 top
R4  40.64,35.56 180 top
R5  45.72,35.56 0 top
R6  17.65,6.35 90 top
R7  5.08,18.67 0 top
R8  16.38,6.35 90 top
R10  34.29,12.83 0 top
R11  34.29,13.84 0 top
R12  34.29,15.37 0 top
R13  34.29,11.3 0 top
R14  34.29,10.29 0 top
R15  15.24,13.97 270 top
R16  36.96,15.24 0 top
R17  14.86,35.43 270 top
R18  10.67,35.43 270 top
R19  36.96,13.97 180 top
R20  37.47,35.69 90 top
R21  36.32,35.69 90 top
R22  11.68,35.43 270 top
RGB  39.37,1.91 90 bottom
S1  16.51,1.78 0 top
S2  34.29,1.78 0 top
SHLD  34.16,5.84 90 bottom
STAT  12.83,1.91 270 bottom
TP1  36.83,2.54 180 bottom
U1  25.4,27.94 90 top
U2  25.4,11.43 0 top
U3  41.27,21.59 90 top
U4  4.95,15.88 0 top
U5  8,15.88 0 top
U6  12.7,21.59 270 top
U7  44.45,29.21 0 top
U8  6.35,29.21 180 top
U9  12.7,15.24 270 top
U10  40.64,13.97 0 top
U$1  [OPENLOG0]  38.1,26.04 0 top
U$2  [RESET0]  16.51,4.06 0 top
U$3  [STAT0]  12.7,5.33 90 top
U$4  [CHG0]  10.79,4.83 90 top
U$5  [CHG0]  10.79,4.83 90 bottom
U$6  [STAT0]  12.7,5.33 90 bottom
U$7  [0_#_BOOT0]  34.29,4.06 0 top
U$8  [IMU0]  41.15,29.21 90 top
U$9  [MAG0]  9.65,29.21 90 top
U$10  [X0]  9.02,34.8 0 top
U$11  [Y0]  7.49,36.2 0 top
U$12  [Z0]  7.49,34.8 0 top
U$13  [X0]  47.12,25.27 0 top
U$14  [Y0]  45.59,26.67 0 top
U$15  [Z0]  45.59,25.27 0 top
U$16  [##RESET##0]  48.77,36.83 0 bottom
U$17  [#0_#_#BOOT##0]  48.77,34.29 0 bottom
U$18  [#36_#_A0#0]  48.77,31.75 0 bottom
U$19  [#39_#_A3#0]  48.77,29.21 0 bottom
U$20  [#35_#_A7#0]  48.77,26.67 0 bottom
U$21  [#17_#_TXD#0]  48.77,24.13 0 bottom
U$22  [#16_#_RXD#0]  48.77,21.59 0 bottom
U$23  [#25#0]  48.77,19.05 0 bottom
U$24  [#26#0]  48.77,16.51 0 bottom
U$25  [#SCL#0]  48.77,13.97 0 bottom
U$26  [#SDA#0]  48.77,11.43 0 bottom
U$27  [#3V3_SW#0]  48.77,8.89 0 bottom
U$28  [#GND#0]  48.77,6.35 0 bottom
U$29  [#GND#1]  2.03,16.51 0 bottom
U$30  [#GND#1]  2.03,21.59 0 bottom
U$31  [#GND#1]  2.03,26.67 0 bottom
U$32  [#BATT#0]  2.03,13.97 0 bottom
U$33  [#5V#0]  2.03,19.05 0 bottom
U$34  [#3V3#0]  2.03,24.13 0 bottom
U$35  [#33#0]  2.03,29.21 0 bottom
U$36  [#POCI_#_19#0]  2.03,31.75 0 bottom
U$37  [#PICO_#_23#0]  2.03,34.29 0 bottom
U$38  [#SCK_#_18#0]  2.03,36.83 0 bottom
U$39  [ESP320]  38.1,24.45 0 top
U$40  [#IMU_INT2#0]  19.81,28.07 0 bottom
U$41  [#MAG_INT#0]  19.81,25.4 0 bottom
U$42  [#35#0]  18.29,27.94 0 bottom
U$43  [#35#0]  18.29,25.4 0 bottom
U$44  [OPENLOG_ESP320]  25.4,21.59 0 bottom
U$45  [#SHLD#0]  34.8,5.84 0 bottom
U$46  [#I�C#0]  36.83,11.49 0 bottom
U$47  [STAT_LED0]  43.18,18.41 0 bottom
U$48  [RGB_LED0]  43.18,17.14 0 bottom
U$49  [RGB0]  39.37,3.81 0 bottom
VIN  8.89,22.86 0 bottom
VIN1  7.62,5.08 0 bottom

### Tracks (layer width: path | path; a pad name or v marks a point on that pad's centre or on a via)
3.3V  (via drill 0.3)
  Top 0.152: C21.1 43.93,33.27 v44.45,33.27 44.97,33.27 C22.1 | U7.P5 43.94,27.56 44.07,27.43 v44.45,27.43 45.34,27.43 45.61,27.71 U7.P8 | v6.35,32.67 6.07,32.38 C23.1 5.58,31.87 4.85,31.14 U8.13 | v6.35,29.21 6.35,28.6 6.1,28.35 U8.2 | U10.14 40.89,15.57 41.06,15.75 v41.4,15.75 | U2.4 24.77,9.75 23.09,11.43 21.59,11.43 20.95,12.06 U2.16 | v38.42,36.77 38.42,36.64 37.97,36.19 R20.2 R21.2
  Top 0.254: U9.14 14.61,14.99 14.73,15.11 15.99,15.11 16.26,14.85 C26.1 C25.1 | v17.4,15.24 17.27,15.11 C25.1 | C25.1 C3.1 | U2.16 20.31,14.23 20.07,14.47 C4.1 C3.1 | v18.16,15.24 18.29,15.11 C3.1
  Top 0.406: v13.97,21.59 14,21.62 U6.5 14,23.34 v13.97,23.37 13.97,23.63 C15.1 C14.1 | v42.04,16.51 v42.04,16.52 41.91,16.64 C28.1 C27.1 v40.64,16.51 | v20.45,23.62 v20.45,21.72 | v27.94,24.89 v27.94,23.37 | C2.1 R22.2 R18.2 10.15,34.93 v9.78,35.31 | R3.2
  Top 0.508: C1.1 C2.1 | U1.2 14.39,33.1 R3.2 | C1.1 R3.2 | C1.1 R17.2 v14.86,33.91 v15.62,33.91
  Route15 0.152: v6.35,32.67 v6.35,29.21 | v44.45,33.27 44.45,30.66 44.83,30.28 44.83,27.81 v44.45,27.43
  Bottom 0.152: I2C.2 v35.69,13.97
  pour Route15 (isolate 0.203): 3.81,0 3.81,2.54 0,2.54 0,38.1 16.26,38.1 16.26,35.81 34.54,35.81 34.54,38.1 50.8,38.1 50.8,0
  cutout Route15: 3.81,26.42 3.81,31.75 8.89,31.75 8.89,26.42
  cutout Route15: 41.91,26.67 41.91,31.75 46.99,31.75 46.99,26.67
3.3V_SW  (via drill 0.3)
  Top 0.406: C18.1 v36.83,16.51 | v38.1,16.51 C19.1 | C20.1 v39.37,16.51 | 34.79,14.6 v34.8,14.61 | 34.79,12.07 v34.8,12.06 | J4.2 44.35,10.95 v44.2,10.79 v44.2,9.91 | 45.22,3.18 45.21,3.17
  Top 0.508: 34.79,14.6 R11.2 R10.2 34.79,12.07 R13.2 R14.2 | R12.2 v34.8,14.61 | J5.2 48.01,7.37 48.01,3.81 47.37,3.17 45.21,3.17 40.28,3.17 | C6.1 C7.1 v37.08,20.32 | v38.1,20.32 C6.1 | U3.5 39.18,20.64 38.73,21.09 C6.1 | J10.2 45.22,3.18 | 40.28,3.17 D2.VCC | C5.1 40.28,4.03 40.28,3.17
  Route15 0.508: 37.47,16.51 v36.83,16.51 35.56,16.51 34.8,15.75 v34.8,14.61 v34.8,12.06 34.42,11.68 31.75,11.68 31.24,12.19 27.05,12.19 v26.29,12.95 v25.53,12.95 | 37.47,16.51 v38.1,16.51 v39.37,16.51 39.37,15.62 v44.2,10.79 | J5.2 47.62,10.79 v44.2,10.79 | v37.08,20.32 37.47,20.32 | 37.47,20.32 37.47,16.51 | v38.1,20.32 37.47,20.32 | v44.2,9.91 v44.2,10.79
  Bottom 0.406: J3.4 25.5,12.98 v25.53,12.95 v26.29,12.95
5V
  Top 0.508: J7.3 2.54,20.32 D6.A
!RESET!  (via drill 0.3)
  Top 0.152: U9.12 v13.2,13.34 v13.21,13.34 13.21,12.45 15.88,9.78 15.88,8.26 16.23,7.9 17.75,7.9 18.39,7.27 18.39,1.85 S1.2 | v37.85,33.02 38.48,33.66 38.48,35.94 39.37,36.83 44.07,36.83 | 44.07,36.83 J8.9 | Q1.3 44.07,36.24 44.07,36.83 | U1.3 16.95,31.62 16,31.62 v15.88,31.5 | v15.24,15.75 15.52,16.03 15.52,20.02 15.21,20.33 15.21,27.68 15.6,28.06 15.6,30.04 15.11,30.52 15.11,31.11 15.49,31.5 v15.88,31.5 | v15.88,31.5 15.88,32.26 15.57,32.57 13.41,32.57 12.84,33.15 R3.1 C31.1
  Bottom 0.152: v37.85,33.02 35.74,33.02 33.46,30.73 28.19,30.73 27.18,31.75 16.13,31.75 v15.88,31.5 | v13.21,13.34 12.18,13.34 11.74,12.9 11.74,12.5 12.02,12.22 14.76,12.22 15.24,12.7 v15.24,15.75
CAP
  Top 0.152: U8.10 6.6,31.87 C24.1
CH340-DTR  (via drill 0.3)
  Top 0.152: R4.2 v39.37,35.56 v39.37,33.02 | Q1.1 43.58,34.91 43.18,35.31 v43.18,35.56 | U2.13 24.77,12.09 25.27,11.58 30.23,11.58 31.85,13.21 31.85,23.51 29.49,25.87 v29.49,29.72
  Bottom 0.152: v39.37,35.56 v43.18,35.56 | v29.49,29.72 29.55,29.77 33.29,29.77 35.77,32.26 38.61,32.26 v39.37,33.02
CH340-RTS  (via drill 0.3)
  Top 0.152: R5.2 v46.99,35.56 | Q1.4 41.62,36.21 41.48,36.35 v41.4,36.35 39.41,36.35 38.83,35.77 38.83,33.27 v38.58,33.02 | v29.97,30.25 29.97,25.91 32.13,23.75 32.13,13.08 30.35,11.3 25.15,11.3 23.5,12.95 U2.14
  Bottom 0.152: v46.99,35.56 46.2,36.35 v41.4,36.35 | v38.58,33.02 38.1,32.54 35.66,32.54 33.37,30.25 v29.97,30.25
CH340-RX  (via drill 0.3)
  Top 0.152: U1.35 33.56,30.48 32.26,30.48 31.75,29.97 31.75,26.75 v31.85,26.65 | v22.86,10.58 23.5,9.94 U2.3 | v23.41,23.62 23.29,23.5 v23.29,18.16
  Bottom 0.152: v31.85,26.65 24.11,26.65 23.37,25.91 23.37,23.67 v23.41,23.62 | v23.29,18.16 21,18.16 20.45,17.61 20.45,14.13 22.48,12.1 22.48,10.96 v22.86,10.58
CH340-TX  (via drill 0.3)
  Top 0.152: U1.34 32.59,29.29 32.23,28.93 v32.23,27.3 | v22.05,10.58 22.05,9.69 22.23,9.52 U2.2 | v22.73,23.62 v22.73,18.67
  Bottom 0.152: v32.23,27.3 24.37,27.3 22.71,25.64 22.71,23.65 v22.73,23.62 | v22.05,10.58 22.05,12.1 20.17,13.98 20.17,17.77 21.07,18.67 v22.73,18.67
D+
  Top 0.305: U2.5 26.04,8.26 25.15,7.37 J1.A6 25.15,5.08 25.4,4.83 26.04,4.83 26.29,5.08 26.29,5.62 26.15,5.76 J1.B6
D-  (via drill 0.3)
  Top 0.305: U2.6 27.3,8.26 26.67,7.62 26.14,7.62 25.65,7.13 J1.A7 25.65,5.4 v25.71,5.4 | J1.B7 24.65,5.5 24.59,5.45 v24.59,5.4
  Bottom 0.305: v25.71,5.4 v24.59,5.4
ESP0/!BOOT!  (via drill 0.3)
  Top 0.152: J8.8 42.29,34.29 | Q1.6 42.26,34.32 42.29,34.29 | v40.13,33.02 40.13,33.78 40.64,34.29 42.29,34.29 | U1.25 v35.01,17.86 35.31,18.16 35.31,30.89 v36.2,31.78 | S2.2 36.24,4.3 v35.46,5.08
  Bottom 0.152: v40.13,33.02 39.09,31.98 36.4,31.98 v36.2,31.78 | v35.46,5.08 35.66,5.28 35.66,6.6 34.75,7.52 34.75,10.26 35.43,10.95 35.43,12.19 35.18,12.45 35.18,14.22 35.43,14.48 35.43,14.73 35.01,15.16 v35.01,17.86
ESP2/DAT0  (via drill 0.3)
  Top 0.152: U9.1 14.47,15.49 14.61,15.62 v14.61,17.25 | U1.24 31.11,17.4 28.07,20.45 v26.42,20.45
  Bottom 0.152: v26.42,20.45 26.29,20.57 20.18,20.57 16.44,16.84 15.02,16.84 v14.61,17.25
ESP4/DAT1  (via drill 0.3)
  Top 0.152: U1.26 32.59,19.13 32.41,18.95 32.41,15.98 v33.02,15.37 R12.1
  Bottom 0.152: J3.8 29.9,15.93 30.48,16.51 31.88,16.51 v33.02,15.37
ESP5/!IMU_CS!  (via drill 0.3)
  Top 0.152: U7.P12 44.95,30.84 v44.93,30.86 | v30.48,33.27 30.48,25.91 32.51,23.88 32.51,23.11 32.69,22.94 U1.29 | R17.1 v14.86,36.83
  Bottom 0.152: v44.93,30.86 44.25,31.54 44.25,32.73 42.46,34.52 38.26,34.52 37.93,34.84 37,34.84 36.67,34.52 35.39,34.52 34.15,33.27 v30.48,33.27 30.23,33.02 17.4,33.02 14.86,35.56 | 14.86,35.56 v14.86,36.83 | IMU_!CS!.1 14.86,35.56
ESP12/DAT2  (via drill 0.3)
  Top 0.152: U9.4 v12.7,18.29 | v16,18.03 16.18,17.86 U1.14
  Bottom 0.152: v16,18.03 15.75,18.29 v12.7,18.29
ESP13/DAT3  (via drill 0.3)
  Top 0.152: U1.16 21.18,16.6 v21.18,17.65 | R14.1 30.36,10.29 v30.1,10.54
  Bottom 0.152: J3.2 23.3,12.14 | v21.18,17.65 21.18,13.87 22.92,12.14 23.3,12.14 | v30.1,10.54 30.05,10.6 24.84,10.6 23.3,12.14
ESP14/CLK  (via drill 0.3)
  Top 0.152: U1.13 19.22,19.13 v19.32,19.04
  Bottom 0.152: v19.32,19.04 19.32,19.32 20.3,20.3 25.43,20.3 26.6,19.12 J3.5
ESP15/CMD  (via drill 0.3)
  Top 0.152: U9.8 10.8,14.99 10.67,14.86 v10.67,13.59 | v24.13,19.18 28.07,19.18 29.84,17.4 U1.23
  Bottom 0.152: v10.67,13.59 10.7,13.56 10.7,12.76 11.79,11.66 14.99,11.66 15.9,12.57 15.9,14.49 20.59,19.18 v24.13,19.18
ESP16/RXD  (via drill 0.3)
  Top 0.152: U1.27 34.75,20.4 v34.83,20.32
  Bottom 0.152: v34.83,20.32 35.31,20.8 35.31,23.1 36.95,24.74 46.38,24.74 J8.3
ESP17/TXD  (via drill 0.3)
  Top 0.152: U1.28 34.75,21.67 v34.83,21.59
  Bottom 0.152: v34.83,21.59 34.83,23.02 36.83,25.02 46.61,25.02 47.5,24.13 J8.4
ESP18/SCK  (via drill 0.3)
  Top 0.152: U8.1 4.64,27.71 v4.58,27.65 | U7.P13 44.45,30.39 v43.97,30.87 | U1.30 32.81,24.21 30.99,26.04 30.99,31.88 v31.75,32.64 | R20.1 v37.47,34.36
  Route15 0.152: v4.58,27.65 4.58,29.98 5.49,30.89 5.49,33.27 4.95,33.81 4.95,34.19 v5.33,34.57
  Bottom 0.152: v43.97,30.87 43.97,32.61 42.34,34.24 37.59,34.24 v37.47,34.36 37.34,34.24 35.63,34.24 34.04,32.64 v31.75,32.64 15.37,32.64 13.82,34.19 6.58,34.19 6.2,34.57 v5.33,34.57 5.31,34.57 3.05,36.83 J6.4
ESP19/POCI  (via drill 0.3)
  Top 0.152: U7.P1 v42.56,29.96 v42.55,29.97 | U1.31 32.18,25.48 31.37,26.29 31.37,30.89 v31.98,31.5 | U8.5 7.22,28.46 v6.99,28.7 | J6.2 6.1,36.58 11.55,36.58 11.68,36.44 R22.1
  Bottom 0.152: v42.55,29.97 42.55,30.91 43.41,31.77 43.41,32.38 42.19,33.6 35.93,33.6 33.83,31.5 v31.98,31.5 27.83,31.5 27.29,32.03 15.09,32.03 13.49,33.63 6.86,33.63 | v6.99,28.7 7.46,29.18 7.46,30 6.83,30.64 6.83,33.6 6.86,33.63 | 6.86,33.63 5.99,33.63 5.79,33.43 5.39,33.43 5.19,33.63 3.15,33.63 J6.2
ESP21/SDA  (via drill 0.3)
  Top 0.152: U1.33 34.62,28.02 34.92,28.32 34.92,31.31 35.87,32.26 39.12,32.26 40.89,30.48 v40.89,23.24 | U10.4 38.78,13.97 v38.73,13.92 37.5,13.92 R19.1 | v4.04,17.78 4.2,17.61 U4.8
  Bottom 0.152: v40.89,23.24 42.9,21.24 42.9,16.36 41.66,15.11 38.56,15.11 38.26,14.8 38.26,14.4 v38.73,13.92 38.73,13.9 38.08,13.24 38.08,12.19 37.57,11.68 36.96,11.68 35.31,10.03 35.31,7.75 36.32,6.73 36.32,4.83 35.31,3.81 34.54,3.81 33.53,2.79 20.41,2.79 16.85,6.35 15.24,6.35 12.7,3.81 5.08,3.81 4.32,4.57 4.32,17.5 v4.04,17.78 | v40.89,23.24
ESP22/SCL  (via drill 0.3)
  Top 0.152: U1.36 35.05,31.83 35.75,32.54 39.23,32.54 41.25,30.52 41.25,23.57 v41.58,23.24 | U10.11 v43.02,13.97 43.02,14.32 43.18,14.48 43.18,15.62 42.8,16 41.83,16 41.6,16.23 41.12,16.23 40.77,15.88 38.73,15.88 38.1,15.24 | 38.1,15.24 R16.2 | 38.1,15.24 38.1,15.28 v38.42,15.59 | v4.72,17.78 4.7,17.77 U4.7
  Bottom 0.152: v41.58,23.24 43.18,21.64 43.18,14.13 v43.02,13.97 | v38.42,15.59 37.8,14.97 37.8,12.31 37.45,11.96 36.84,11.96 35.03,10.15 35.03,7.63 35.94,6.72 35.94,4.85 35.18,4.09 34.43,4.09 33.41,3.07 20.56,3.07 17.01,6.63 15.12,6.63 12.58,4.09 5.2,4.09 4.6,4.69 4.6,17.66 v4.72,17.78
ESP23/PICO  (via drill 0.3)
  Top 0.152: U7.P14 43.3,30.86 v43.18,30.86 | v32.26,32.13 32.26,32.74 32.62,33.1 U1.37 35.89,33.1 36.32,33.54 R21.1 | U8.16 5.53,28.47 v5.74,28.68
  Route15 0.152: v5.74,28.68 5.24,29.18 5.24,30 5.87,30.64 5.87,33.63 v5.59,33.91
  Bottom 0.152: v43.18,30.86 43.69,31.37 43.69,32.49 42.3,33.88 35.79,33.88 34.04,32.13 v32.26,32.13 27.69,32.13 27.46,32.36 15.25,32.36 13.7,33.91 v5.59,33.91 2.92,33.91 2.54,34.29 J6.3
ESP25/LED  (via drill 0.3)
  Top 0.152: v15.97,23.21 16.89,23.21 U1.10 | R6.2 17.65,7.37 17.4,7.62 16,7.62 14.25,5.87 v11.79,5.87 v11.78,5.87
  Bottom 0.152: v11.78,5.87 11.29,5.87 10.61,6.55 9.48,6.55 8.18,7.85 8.18,11.59 9.53,12.94 9.53,21.97 11.68,24.13 15.06,24.13 v15.97,23.21 16.89,24.13 20.95,24.13 22.23,22.86 33.02,22.86 34.35,21.53 34.35,20.12 34.63,19.84 35.02,19.84 35.59,20.4 35.59,22.89 37.16,24.46 46.27,24.46 48.26,22.46 48.26,20.32 J8.2
ESP26/RGBLED  (via drill 0.3)
  Top 0.152: v18.41,21.72 18.37,21.67 U1.11
  Bottom 0.152: v18.41,21.72 18.41,22.99 18.57,23.14 21.55,23.14 22.11,22.58 32.9,22.58 34.07,21.42 34.07,20 34.51,19.56 35.14,19.56 35.87,20.29 35.87,22.77 37.28,24.18 46.15,24.18 47.98,22.35 47.98,18.06 J8.1 47.32,14.3 47.32,8.26 46.85,7.78 44.74,7.78 41.53,4.57 41.53,2.79 41.16,2.43 RGB.2
ESP27/!MAG_CS!  (via drill 0.3)
  Top 0.152: U8.4 7.47,27.71 7.75,27.43 v7.75,27.3 | U1.12 16.16,20.4 15.7,20.86 v15.7,21.59 15.7,22.66 15.49,22.86 15.49,27.56 15.88,27.94 15.88,30.56 v15.65,30.79 | R18.1 10.66,35.94 8.26,35.94 7.62,35.31 v7.62,33.15
  Bottom 0.152: v7.75,27.3 7.75,30.11 7.11,30.75 7.11,32.64 v7.62,33.15 13.29,33.15 v15.65,30.79 | v15.7,21.59 15.24,21.14 MAG_!CS!.1
ESP32/PWREN  (via drill 0.3)
  Top 0.152: U1.8 18.46,25.48 19.05,24.89 v19.05,23.62 | U9.11 12.7,12.23 12.19,11.73 11.01,11.73 v10.67,12.06
  Bottom 0.152: v19.05,23.62 17.27,23.62 16.38,22.73 15.78,22.73 14.66,23.85 11.8,23.85 9.8,21.86 9.8,12.93 v10.67,12.06
ESP33  (via drill 0.3)
  Top 0.152: U1.9 16.05,24.21 v15.97,24.13
  Bottom 0.152: v15.97,24.13 15.39,24.71 4.48,24.71 3.05,26.15 3.05,27.4 1.27,29.18 J6.1
ESP34/IMU_INT1  (via drill 0.3)
  Top 0.152: U7.P4 v42.56,28.46 v42.55,28.45 | v19.56,33.91 19.56,30.23 20.19,29.59 20.19,28.96 19.26,28.02 U1.6
  Bottom 0.152: v42.55,28.45 45.09,28.45 45.54,28.9 45.54,33.12 43.86,34.8 38.37,34.8 38.04,35.12 36.89,35.12 36.56,34.8 31.24,34.8 29.84,33.4 20.07,33.4 v19.56,33.91 18.95,33.3 17.52,33.3 15.37,35.45 15.37,37.08 14.99,37.47 12.06,37.47 11.43,36.83 IMU_INT1.1
ESP35/A7  (via drill 0.3)
  Top 0.152: v19.05,26.67 17.24,26.67 U1.7
  Bottom 0.152: v19.05,26.67 20.32,26.67 20.83,27.18 20.83,29.51 21.77,30.45 26.19,30.45 27.99,28.65 33.93,28.65 36.85,25.73 47.32,25.73 48.26,26.67 J8.5
  Bottom 0.203: IMU_INT2.2 18.64,27.08 v19.05,26.67 18.64,26.26 MAG_INT.2
ESP36/A0  (via drill 0.3)
  Top 0.152: v18.54,30.48 18.46,30.56 U1.4
  Bottom 0.152: J8.7 47.24,29.46 47.24,26.54 46.99,26.29 37.08,26.29 34.16,29.21 28.45,29.21 26.57,31.09 19.15,31.09 v18.54,30.48
ESP39/A3  (via drill 0.3)
  Top 0.152: U1.5 18.11,29.29 v18.54,29.72
  Bottom 0.152: J8.6 47.52,27.2 47.52,26.43 47.11,26.01 36.97,26.01 34.05,28.93 28.2,28.93 26.33,30.81 19.63,30.81 v18.54,29.72
GND  (via drill 0.3)
  Top 0.152: U4.6 5.2,16.12 U4.9 | U4.1 4.2,15.38 4.7,15.88 U4.9 | U4.4 5.7,15.38 5.21,15.88 U4.9 | U7.P3 43.97,28.96 v44.22,29.21 | U7.P2 43.97,29.46 v44.22,29.21 | v8.89,32.64 8.64,32.38 C24.2 7.1,31.36 U8.9 7.1,29.83 v6.99,29.72 6.48,29.72 6.1,30.1 U8.11 | C23.2 4.06,32.38 v3.81,32.64 | U9.EPAD 12.45,15.49 U9.7 10.93,15.49 10.67,15.75 v10.67,15.88 | U7.P7 44.95,28.96 44.7,29.21 v44.22,29.21 | U7.P6 44.45,28.98 v44.22,29.21 | U10.6 39.89,12.97 40.64,13.72 U10.EPAD 40.64,14.22 41.39,14.97 U10.13
  Top 0.254: J1.GND2 28.62,5.84 28.92,5.55 28.92,4.79 v27.94,3.81 | J1.GND 22.18,5.84 21.88,5.55 21.88,4.79 v22.86,3.81 | C26.2 16.26,12.95 v16.51,12.7 | U10.7 v40.39,11.43 | U10.13 42.14,15.37 v42.67,15.37
  Top 0.406: v8,15.88 U5.2
  Bottom 0.152: v28.45,29.97 26.95,31.47 17.5,31.47 16,29.97 16,27.43 14.73,26.16 v13.34,26.16 | v35.84,25.4 v48.29,25.4
  Bottom 0.305: SHLD.1 v34.16,4.57
  other vias: 31.11,1.91 31.11,4.45 37.47,1.4 7.11,12.7 7.11,8.89 7.11,10.79 15.75,2.16 18.54,34.29 12.83,36.83 13.84,36.83 19.3,5.08 19.3,12.7 20.95,9.91 12.7,21.59 13.97,19.18 12.06,26.16 10.79,26.16 41.94,33.02 46.99,33.02 31.75,34.29 22.1,29.97 25.78,29.97 25.78,24 22.1,24 23.88,29.97 24.13,24 45.49,22.86 44.48,22.86 46.51,22.86 41.05,21.59 39.37,19.05 40.64,19.05 41.91,19.05 36.7,19.05 38.23,19.05 2.54,30.48 17.78,12.7 10.35,21.59 7.75,20.83 43.12,5.08 44.2,3.94 45.59,9.91 46.61,8.64 37.11,22.86 38.1,22.86 38.1,4.45 19.68,17.53 27.69,13.21 32.77,12.45 30.48,20.32 48.29,35.56 3.56,35.56 25.4,17.78 19.68,1.91 18.29,8.64 4.57,22.99 14.48,14.35 5.65,35.37 35.56,36.96 8.51,18.29 22.86,34.29 26.67,34.29
  pour Top (isolate 0.203): 3.81,0 3.81,2.54 0,2.54 0,38.1 16.26,38.1 16.26,35.81 34.54,35.81 34.54,38.1 50.8,38.1 50.8,0
  pour Bottom (isolate 0.203): 3.81,0 3.81,2.54 0,2.54 0,38.1 16.26,38.1 16.26,35.81 34.54,35.81 34.54,38.1 50.8,38.1 50.8,0
  pour Route2 (isolate 0.203): 3.81,0 3.81,2.54 0,2.54 0,38.1 16.26,38.1 16.26,35.81 34.54,35.81 34.54,38.1 50.8,38.1 50.8,0
  cutout Top: 3.81,31.75 3.81,26.42 8.89,26.42 8.89,31.75
  cutout Bottom: 3.81,26.42 3.81,31.75 8.89,31.75 8.89,26.42
  cutout Route2: 45.72,31.75 46.99,31.75 46.99,26.67 41.91,26.67 41.91,31.75 43.18,31.75 43.18,31.62 42.04,31.62 42.04,26.8 46.86,26.8 46.86,31.62 45.72,31.62
  cutout Bottom: 41.91,26.67 41.91,31.75 46.99,31.75 46.99,26.67
  cutout Top: 41.91,31.75 41.91,26.67 46.99,26.67 46.99,31.75
  cutout Route2: 5.08,31.75 3.81,31.75 3.81,26.42 8.89,26.42 8.89,31.75 7.62,31.75 7.62,31.62 8.76,31.62 8.76,26.54 3.94,26.54 3.94,31.62 5.08,31.62
IMU_INT2  (via drill 0.3)
  Top 0.152: U7.P9 46.1,28.96 46.35,28.7 v46.35,28.32 | v19.94,34.62 19.56,34.62 19.05,34.11 19.05,29.72 v19.43,29.34
  Bottom 0.152: v46.35,28.32 45.82,28.86 45.82,33.23 43.98,35.08 38.49,35.08 38.16,35.4 36.77,35.4 36.44,35.08 31.06,35.08 29.72,33.73 20.83,33.73 v19.94,34.62
  Bottom 0.203: IMU_INT2.1 19.46,29.31 v19.43,29.34
MAG_INT  (via drill 0.3)
  Top 0.152: U8.15 5.35,28.97 5.71,29.34 v5.71,29.72
  Bottom 0.152: v5.71,29.72 5.71,32.33 4.83,33.22 3.59,33.22 3.33,32.97 3.33,26.26 4.6,24.99 15.79,24.99 16.37,24.41 19.3,24.41 19.46,24.56 MAG_INT.1
N$1
  Top 0.152: J1.B5 27.15,7.08 27.3,7.24 31.36,7.24 R1.2
N$2
  Top 0.152: J1.A5 24.15,7.09 24,7.24 19.44,7.24 R2.2
N$4
  Top 0.152: Q1.2 R5.1
N$5
  Top 0.152: Q1.5 R4.1
N$6  (via drill 0.3)
  Top 0.152: R6.1 17.78,5.72 v17.78,4.7
  Bottom 0.152: STAT.2 15.73,1.38 16.13,1.78 17.02,1.78 17.78,2.54 v17.78,4.7
N$7  (via drill 0.3)
  Top 0.152: D2.DO 37.73,3.17 v37.72,3.17
  Bottom 0.152: TP1.1 37.08,2.54 v37.72,3.17
N$8  (via drill 0.3)
  Top 0.152: v9.4,1.14 9.4,1.39 D3.A
  Bottom 0.152: CHG.1 9.64,1.38 v9.4,1.14
N$9
  Top 0.152: R8.1 15.37,5.85 14.22,4.7 12.19,4.7 11.81,4.32 11.81,2.04 D3.C
N$10  (via drill 0.3)
  Top 0.152: v7.11,15.88 7.05,15.81 U5.1 | v11.81,5.08 14.11,5.08 15.88,6.85 R8.2
  Bottom 0.152: v7.11,15.88 7.11,15.24 7.62,14.73 7.62,7.62 8.89,6.35 | v11.81,5.08 10.16,5.08 8.89,6.35 | VIN1.1 8.89,6.35
N$11
  Top 0.152: U5.5 6.57,17.18 5.59,18.16 R7.2
N$12  (via drill 0.3)
  Top 0.152: v41.27,1.4 41.23,1.35 D2.DI
  Bottom 0.152: RGB.1 41.26,1.38 v41.27,1.4
N$13  (via drill 0.3)
  Top 0.152: D1.A 13.03,3.12 v13.78,3.12
  Bottom 0.152: v13.78,3.12 13.09,2.43 STAT.1
N$16  (via drill 0.3)
  Top 0.152: R16.1 v35.69,15.24
  Bottom 0.152: v35.69,15.24 35.92,15.01 I2C.1
N$17  (via drill 0.3)
  Top 0.152: R19.2 36.46,13.47 v35.69,12.7
  Bottom 0.152: v35.69,12.7 35.92,12.93 I2C.3
PWREN  (via drill 0.3)
  Top 0.152: U10.12 42.41,14.47 v42.55,14.61 | U9.13 13.7,13.46 | 13.7,13.46 13.7,12.71 v13.69,12.7 | R15.2 13.71,13.47 13.7,13.46 | v12.22,12.7 12.22,14.12 U9.10 | U9.5 12.2,16.88 v11.94,17.14 11.7,16.91 U9.6 | U3.3 43.37,22.54 v43.69,22.86 | v41.15,19.68 v43.66,19.68 | v38.86,12.7 38.86,13.34 39,13.47 U10.5
  Bottom 0.152: v42.55,14.61 42.04,14.1 | 42.04,14.1 40.64,12.7 v38.86,12.7 | v12.22,12.7 v13.69,12.7 13.69,15.39 13.27,15.81 | 13.27,15.81 v11.94,17.14 11.94,18.2 12.5,18.77 12.9,18.77 13.1,18.57 16.99,18.57 18.57,20.15 18.57,20.9 18.88,21.21 26.81,21.21 28.97,19.05 35.94,19.05 36.58,19.68 v41.15,19.68 | v43.69,22.86 43.5,22.67 43.5,19.68 | 43.5,19.68 43.5,13.77 43.22,13.49 42.64,13.49 42.04,14.1 | PWREN.1 13.27,15.81 | v43.66,19.68 43.5,19.68
QWIIC_SCL  (via drill 0.3)
  Top 0.152: J5.4 48.51,12.95 J4.4 43.31,12.95 42.79,13.47 U10.10 | J10.4 47.22,6.12 47.12,6.22 v47.12,7.24
  Bottom 0.152: v47.12,7.24 47.6,7.72 47.6,12.04 J5.4
QWIIC_SDA  (via drill 0.3)
  Top 0.152: J5.3 48.26,11.43 47.74,11.95 J4.3 45.58,11.95 v45.09,12.45 | J10.3 46.22,6.04 46.04,6.22 v46.04,7.24 | U10.3 38.87,14.47 v38.73,14.61
  Bottom 0.152: v46.04,7.24 46.04,6.73 46.42,6.35 47.37,6.35 47.88,6.86 47.88,9.78 J5.3 | v38.73,14.61 39.24,14.1 39.24,13.46 39.1,13.32 38.67,13.32 38.35,13 38.35,12.53 38.82,12.06 44.7,12.06 v45.09,12.45
SD_CMD  (via drill 0.3)
  Top 0.152: U9.9 11.7,13.48 11.43,13.21 v11.3,13.21 | R10.1 33.66,12.95 32.52,12.95 31.11,11.55 v31.11,11.2
  Bottom 0.152: v11.3,13.21 11.3,12.54 11.9,11.94 14.88,11.94 15.62,12.69 15.62,14.61 20.67,19.66 24.41,19.66 24.65,19.42 24.65,14.87 J3.3 24.4,12.43 25.25,11.59 30.73,11.59 v31.11,11.2
SD_DAT0  (via drill 0.3)
  Top 0.152: U9.2 13.7,17.34 v13.74,17.38 | R11.1 33.79,14.6 v33.78,14.61
  Bottom 0.152: v13.74,17.38 14.09,17.73 15.23,17.73 15.72,17.24 16.45,17.24 20.14,20.93 26.7,20.93 28.8,18.83 28.8,16.76 | 28.8,16.76 J3.7 | v33.78,14.61 33.78,15.28 32.28,16.79 28.82,16.79 28.8,16.76
SD_DAT2  (via drill 0.3)
  Top 0.152: U9.3 v13.2,17.8 v13.21,17.81 | v19.05,20.7 v22.1,17.65 | R13.1 32,11.3 31.43,10.72 30.68,10.72 30.38,11.02 24.78,11.02 22.89,12.91 v22.82,12.91
  Bottom 0.152: v13.21,17.81 13.41,18.01 15.35,18.01 15.84,17.52 16.34,17.52 19.05,20.23 v19.05,20.7 | v22.1,17.65 22.2,17.55 J3.1 22.2,13.52 22.8,12.91 v22.82,12.91
SHIELD  (via drill 0.3)
  Route2 0.305: J1.SHLD1 21.08,5.18 20.57,4.66 20.57,3.21 21.08,2.7 J1.SHLD3 J1.SHLD4 29.72,2.7 30.23,3.21 30.23,4.66 29.72,5.17 J1.SHLD2 32.87,5.82 v34.16,7.11
  Bottom 0.305: v34.16,7.11 SHLD.2
V_BATT
  Top 0.305: U4.2 4.7,13.97 | U4.3 5.2,13.97
  Top 0.406: 4.2,13.97 4.19,13.97 4.08,13.86 | 4.7,13.97
  Top 0.508: 4.19,13.97 3.05,13.97 | 3.05,13.97 J7.1 | 4.2,13.97 4.7,13.97 5.2,13.97 | J2.2 4.08,13.86 | 4.7,13.97 5.34,13.97 5.85,13.46 8.38,13.46 8.95,14.03 U5.3 9.49,14.57 9.91,14.99 9.91,18.53 C11.1 C30.1 9.39,20.52 9.02,20.89 8.61,20.89 8.26,21.25 D4.A | C13.1 3.05,13.97
V_USB  (via drill 0.3)
  Top 0.406: v23.5,4.45 23.5,5.33 22.95,5.88 J1.VBUS1 | v27.3,4.45 27.3,5.33 27.85,5.88 J1.VBUS2
  Top 0.508: v3.17,22.86 3.17,23.24 3.29,23.36 D5.A 3.29,25.03 v3.17,25.15 | v19.56,11.18 19.22,11.52 D7.2 17.23,11.52 v16.89,11.18
  Route15 0.711: v3.17,25.15 v3.17,22.86 3.17,14.61 3.81,13.97 7.62,13.97 8.89,12.7 8.89,11.94 9.65,11.18 v16.89,11.18 v19.56,11.18 21.2,11.18 21.48,11.46 23.08,11.46 24.13,10.41 24.13,7.62 23.5,6.99 v23.5,4.45 v27.3,4.45
VIN  (via drill 0.3)
  Top 0.152: U5.4 8.95,15.94 v8.89,15.88 | v9.4,2.54 9.78,2.92 9.78,5.81 v10.03,6.07
  Top 0.508: C10.1 v46.48,20.32 45.47,20.32 | 45.47,20.32 v44.45,20.32 C9.1 43.95,21.09 43.5,20.64 U3.1 | C8.1 45.47,20.32 | v12.7,22.48 12.64,22.54 U6.1 | U6.3 12.64,20.64 v12.7,20.7 | C17.1 11.4,19.98 U6.3 | U5.4 8.1,17.18 7.87,17.4 7.87,17.91 7.24,18.54 C12.1 6.47,19.06 5.59,19.93 D6.C 5.58,20.34 C29.1 v5.58,23 5.58,24.11 D5.C 6.73,24.13 6.86,24 8.25,24 D4.C 9.53,24.01 9.79,24.27 C16.1 10.79,23.75 11.4,23.14 U6.1 | U6.1 10.22,22.54 9.69,22.01 9.69,21.3 10.35,20.64 U6.3
  Route15 0.508: v46.48,20.32 v44.45,20.32 44.07,20.32 43.69,20.7 40.77,20.7 39.5,21.97 36.45,21.97 34.29,24.13 27.43,24.13 26.92,23.62 26.92,22.23 26.54,21.84 21.72,21.84 21.08,22.48 v12.7,22.48 12.19,22.48 11.94,22.23 11.94,20.95 12.19,20.7 v12.7,20.7
  Bottom 0.152: v8.89,15.88 8.89,12.7 7.9,11.71 7.9,7.74 9.57,6.07 v10.03,6.07 | v9.4,2.54 10.68,2.54 CHG.2 | VIN.1 5.72,22.86 v5.58,23

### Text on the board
Route2: 2
Route15: 3
Bottom: v10
Measures: Dimensions / In Inches
tDocu: 4-Layers / 1.6mm Thickness / 1oz Copper / Lead-Free HASL Finish / Red Solder Resist / White Silkscreen | Paul Clark

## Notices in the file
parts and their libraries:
SparkFun-Aesthetics: Licensing: Creative Commons ShareAlike 4.0 International - https://creativecommons.org/licenses/by-sa/4.0
SparkFun-Aesthetics: Released under the Creative Commons Attribution Share-Alike 4.0 License
SparkFun-Aesthetics: https://creativecommons.org/licenses/by-sa/4.0
